(* Logix 5000 Rung export; software revision 16.04 *)

MODULES
   Local : vendor None type None code None
   AFC : vendor None type None code None
END_MODULES

TYPE AFC_ModbusPassThruIn :   // Modbus pass through input
STRUCT
   BID : INT;   // Calculated by ladder logic
   MessagePresent : BOOL;   // Message present in the response block
   Function_BitWrite : BOOL;   // Function bit write
   OverflowError : BOOL;   // Overflow error flag
   ModbusAddress : INT;   // Destination modbus address
   RegisterCount : INT;   // Number of elements associated to command
   ReadData_Word : INT[125];   // Contains received data for word commands
   ReadData_Bit : BOOL[2016];   // Contains received data for bit commands
END_STRUCT
END_TYPE

TYPE AFC_Prove_Config :   // Controls (configuration settings) associated to the prover
STRUCT
   Enable : AFC_Prove_Config_Enable;   // Controls at enable
   Accept : AFC_Prove_Config_Accept;   // Controls at accept
END_STRUCT
END_TYPE

TYPE AFC_Prove_Phase_Bitmap :   // AFC prove phase bitmap
STRUCT
   Not_Selected : BOOL;   // Not selected
   Active : BOOL;   // Active, not counting
   Counting_Past_1st_Switch : BOOL;   // Counting past 1st switch for Udir and forward leg for Bdir)
   Past_2nd_Switch_Fwd_Leg : BOOL;   // Past 2nd switch forward leg (bidirectional only)
   Past_1st_Swith_Ret_Leg : BOOL;   // Past 1st switch return leg (bidirectional only)
   Run_Complete : BOOL;   // Run complete. past 2nd switch.
END_STRUCT
END_TYPE

TYPE AFC :   // Main user defined data type
STRUCT
   Meters : AFC_Meters[16];   // Stores meter process variables, results, analysis (gas) and module profile
   MeterSignals : AFC_Meter_Reset;   // Sets meter signals (write archive, reset accumulator and select stream)
   ModbusGateway : AFC_Modbus;   // Reads and write data between processor and module modbus table
   ModbusMaster : AFC_ModbusMaster;   // Setup modbus master commands to be sent to remote slaves (through Port 3)
   ModbusPassThru : AFC_ModbusPassThru;   // Modbus pass-thru data
   Prove : AFC_Prove;   // Proving implementation (only firmware 2.07.000 or later)
   Flags : AFC_Flag;   // Wallclock update commands
   EnableMeter : AFC_Meter;   // Enable meters (this action can also be performed through AFC Manager)
   DisableMeter : AFC_Meter;   // Disable meters (this action can also be performed through AFC Manager)
   EnableStatus : AFC_Meter;   // Meter current status (0=disabled, 1=enabled)
   Site_Status : AFC_Site_Status;   // Site status
   Site_Alarms : AFC_Site_Alarms;   // Site Alarms
   CycleCounter : INT;   // Reflects current block ID calculated by ladder to be sent to the module
   inputbuffer : INT[250];   // Input buffer contains the complete block to be copied from the module
   outputbuffer : INT[248];   // Output buffer contains data the complete block to be copied to the module
   clockstructure : AFC_Time;   // Stores clock information
   Util : AFC_Util;   // Convenience variables used by ladder logic
END_STRUCT
END_TYPE

TYPE AFC_ModbusGateway :   // Modbus gateway complete data structure
STRUCT
   Config : AFC_ModbusConfig;   // Config data to be entered by the user.
   BOD : INT;   // Block ID automatically generated by ladder
   WriteData : INT[200];   // Contains modbus data written to the module (write commands)
   BID : INT;   // Block ID automatically generated by ladder
   ReadData : INT[200];   // Contains modbus data read from the module (read commands)
END_STRUCT
END_TYPE

TYPE AFC_Meter_Variables :   // Meter process variables from processor to the module.
STRUCT
   BID : INT;   // Block ID associated to meter process variable block (from processor to the module)
   DifferentialGas : AFC_Meter_Differential_Gas_Output;   // Differential meter and gas product
   DifferentialLiquid : AFC_Meter_Differential_Liquid_Output;   // Differential meter and liquid product
   LinearGas : AFC_Meter_Linear_Gas_Output;   // Linear meter and gas product
   LinearLiquid : AFC_Meter_Linear_Liquid_Output;   // Linear meter and liquid product
END_STRUCT
END_TYPE

TYPE AFC_Components_Low :   // Low precision gas component analysis
STRUCT
   C1 : INT;   // Methane
   N2 : INT;   // Nitrogen
   CO2 : INT;   // Carbon dioxide
   C2 : INT;   // Ethane
   C3 : INT;   // Propane
   H20 : INT;   // Water
   H2S : INT;   // Hydrogen sulphide
   H2 : INT;   // Hydrogen
   CO : INT;   // Carbon monoxide
   O2 : INT;   // Oxygen
   IC4 : INT;   // Iso-butane
   NC4 : INT;   // Normal butane
   IC5 : INT;   // Iso-pentane
   NC5 : INT;   // Normal pentane
   C6 : INT;   // Hexane
   C7 : INT;   // Heptane
   C8 : INT;   // Octane
   C9 : INT;   // Nonane
   C10 : INT;   // Decane
   He : INT;   // Helium
   Ar : INT;   // Argon
   NeoC5 : INT;   // Not used
   Ux_User1 : INT;   // Not used
   Uy_User2 : INT;   // Not used
END_STRUCT
END_TYPE

TYPE AFC_Modbus :   // Modbus Gateway data structure. Select the number of commands to be used (1 to 10). O will disable this funcionality.
STRUCT
   CommandCount : INT;   // Defines the number of Modbus Gateway Blocks to be used (1 to 10). Set to 0 to disable the feature.
   Command : AFC_ModbusGateway[10];   // Modbus gateway commands - contains setup and modbus data
END_STRUCT
END_TYPE

TYPE AFC_Status :   // General meter configuration profile
STRUCT
   MeterType : BOOL;   // 0=Differential, 1=Linear
   ProductGroup : BOOL;   // 0=Gas, 1=Liquid
   SelectedStream : INT;   // Selected Stream (1 through 4). Only supported for firmware version 2.05.000 or later
END_STRUCT
END_TYPE

TYPE AFC_Prove_Process :   // Prove process output from processor to the module
STRUCT
   Sequencing : AFC_Prove_Sequencing;   // Prover sequencing
   Temperature : REAL;   // Temperature for Single Probe provers. And Inlet Temperature for Dual Probe Provers.
   Outlet_Temperature : REAL;   // Outlet Temperature for Provers with Dual Probes.
   Switch_Bar_Temperature : REAL;   // Switch bar temperature
   Pressure : REAL;   // Pressure for Single Probe provers. And Inlet Pressure for Dual Probe Provers.
   Outlet_Pressure : REAL;   // Outlet Pressure for Provers with Dual Probes.
   Prover_Density : REAL;   // Prover density
END_STRUCT
END_TYPE

TYPE AFC_Analysis_Status :   // Contains stream configuration information concerning high/low precision.
STRUCT
   Update : BOOL;   // Trigger update of analysis status
   Stream_Precision : SINT[4];   // Stream Precision ( 1 = Low, 2 = High)
   Slot_In_Stream : SINT[4];   // Slot number associated to each stream (0-BASED) Ex: (Slot_In_Stream[0] = 1 means stream 1 is set for slot 2)
   Slot_Precision : SINT[4];   // Precision of each slot (0-BASED) (2=high precision/first slot, 1=low precision,0=high precision/second slot)
END_STRUCT
END_TYPE

TYPE AFC_Meter_Differential_Gas_Output :   // Process Variables for differential meter with gas product
STRUCT
   Temperature : REAL;   // Temperature
   Pressure : REAL;   // Static pressure
   Differential_Pressure : REAL;   // Differential pressure if Primary Input = Differential pressure OR Flow Rate if Primary Input = Flow rate
END_STRUCT
END_TYPE

TYPE AFC_Site_Status :   // Site status bits - contains general information about the module - not meter specific
STRUCT
   AFC_ACTIVE : BOOL;   // AFC active
   Checksum_Alarms : BOOL;   // Checkum alarm active
   reserved2 : BOOL;
   reserved3 : BOOL;
   PLC_HALTED : BOOL;   // PLC in program mode or missing
   Cfg_changed : BOOL;   // Configuration changed
   Powerup : BOOL;   // Module powered up
   ColdStart : BOOL;   // Module performed cold start (BBRAM initialized)
   HardPassword : BOOL;   // Hard password selected
   reserved9 : BOOL;
   reserved10 : BOOL;
   reserved11 : BOOL;
   reserved12 : BOOL;
   reserved13 : BOOL;
   reserved14 : BOOL;
   reserved15 : BOOL;
END_STRUCT
END_TYPE

TYPE AFC_Meter_Linear_Liquid_Output :   // Process Variables for linear meter with liquid product
STRUCT
   Water_Percent : INT;   // Water (%)
   Temperature : REAL;   // Temperature
   Pressure : REAL;   // Pressure
   Meter_Pulses : DINT;   // Meter pulses
   Density : REAL;   // Density
   Pulse_Frequency : REAL;   // Pulse frequency (Hz)
END_STRUCT
END_TYPE

TYPE AFC_Prove_Pulse_Count :   // Values to be supplied at the end of the pass/run
STRUCT
   Meter : DINT;   // Meter pulse count
   Master_Meter : DINT;   // Master meter pulse count
END_STRUCT
END_TYPE

TYPE AFC_Prove_Run_Results :   // Run results of the prove. Copied from the module to the pocessor
STRUCT
   Count_Attempted : INT;   // Run count attempted
   Count_Completed : INT;   // Run count completed
   Count_Selected : INT;   // Run count selected
   Runs_Selected : INT;   // Bit Mapped Runs selected for calculations from completed runs
   New_Meter_Factor : REAL;   // New meter factor
   Change_In_Meter_Factor : REAL;   // Change in meter factor
END_STRUCT
END_TYPE

TYPE AFC_ModbusMasterSwap :   // Modbus master swap words/ swap bytes
STRUCT
   Swap_Words : BOOL;   // Swap words
   Swap_Bytes : BOOL;   // Swap bytes
END_STRUCT
END_TYPE

TYPE AFC_Prove_Config_Enable :   // Prove controls at enable
STRUCT
   Meter_Number : INT;   // Meter number requested (1-16)
   Auto_Accept_Prove : BOOL;   // Auto-accept the prove
   Auto_Continue_Prove : BOOL;   // Auto-continue the prove
END_STRUCT
END_TYPE

TYPE AFC_ModbusMasterIn :   // Modbus master input tag.
STRUCT
   BID : INT;   // Block id associated to modbus master request
   TransactionNumber : INT;   // Transaction number associated to modbus command index
   ErrorCode : INT;   // Error code associated to modbus master command
   Pending : BOOL;   // Pending modbus master command - waiting for modbus response
   ReadData : INT[100];   // Data read fro mremote slave device
END_STRUCT
END_TYPE

TYPE AFC_Prove_Input :   // AFC Prove input block
STRUCT
   Config : AFC_Prove_Input_Config;   // AFC prover input configuration
   Status : AFC_Prove_Status;   // AFC prover status
   Error_Code : INT;   // Prove error code
   Prove_controls_Echo : INT;   // AFC module Echos the state of the Prove Controls
   Requested_Meter_Echo : INT;   // AFC module Echos the Meter number requested
   Requested_Curve_Point_Echo : INT;   // AFC module Echos the requested Curve Point
   Run_Results : AFC_Prove_Run_Results;   // Prove and run results
   Prove_Enabled : BOOL;   // ON if prove is enabled. This flag is coped from inputbuffer[247]
END_STRUCT
END_TYPE

TYPE AFC_Util :   // Used for internal ladder logic usage. These values must not be changed by user application.
STRUCT
   MeterIndex1 : INT;   // Meter index for process variable calculation
   Offset1 : INT;   // Offset for meter process calculation
   MeterIndex2 : INT;   // Meter index for calculation results
   Offset2 : INT;   // Offset for calculation results
   SignalsTimer : TIMER;   // Signals timer
   IndexOut : INT;   // Index output
   IndexIn : INT;   // Index input
   CycleCounterRollover : INT;   // Rollover value for cycle counter for block ID calculation
   LongCount : INT;   // Long count for modbus master command
   LastRegularBlockID : INT;   // Rollover block ID
   Current_meter : SINT;   // Current meter number analysis update
   MaskedStream : INT;   // Masked stream
   AnalysisMeterNumber : INT;   // Analysis meter number
   AnalysisBID : INT;   // Analysis block ID
   AnalysisStreamMasked : INT;   // Analysis stream masked information
   v206orLater : INT;   // indicates if the meter is 2.06 or later so the module supports high precision analysis
   AnalysisHighPrecisionBOD : INT;   // Analysis high precision number
   Firmware_Version : SINT[2];   // Firmware version number
   Firmware_Revision : INT;   // firmware revision number
   AnalysisHMeter : INT;   // Meter associated to molar high precision
   SlotPrecision : SINT[4];   // Slot precision number for stream precision calculation
   SlotInStream : DINT[4];   // Slot number for stream X
   PowerUp_HighAnalysis : BOOL;   // Request high analysis block upon power up
   Meter_HighAnalysis : INT;   // Meter number for high precision analysis
   TempSlotInStream : SINT;   // Used to calculate stream precision based on slot precision
   AnalysisHighPrecisionBID : INT[16];   // High precision block ID
   AnalysisHighPrecisionBID_Update : INT;   // molar block id update
   Reinitialize_Timer : TIMER;   // Timer to initialize block ID if freezes
   Prover_Phase : INT;   // Prover phase integer word to assemble all bits
   Prover_Signals : INT;   // Prover signals integer word to assemble all bits
   Prover_Controls : INT;   // Prover control word to assemble all bits
END_STRUCT
END_TYPE

TYPE AFC_Time :   // AFC time format used for walclock update
STRUCT
   Year : DINT;   // Year
   Month : DINT;   // Month
   Day : DINT;   // Day
   Hour : DINT;   // Hour
   Minute : DINT;   // Minute
   second : DINT;   // Seconds
   msec : DINT;   // Milliseconds
END_STRUCT
END_TYPE

TYPE AFC_ModbusPassThru :   // AFC modbus pass through controller tag
STRUCT
   Output : AFC_ModbusPassThruOut;   // Values to be transferred from processor to the module
   Input : AFC_ModbusPassThruIn;   // Values to be transferred from module to processor
END_STRUCT
END_TYPE

TYPE AFC_Meter_Results :   // AFC meter results calculated by the module to the processor
STRUCT
   BID : INT;   // Block ID associated to calculation results
   Alarms : INT;   // Meter alarms
   DifferentialGas : AFC_Meter_Differential_Gas_Input;   // Differential meter / product gas
   DifferentialLiquid : AFC_Meter_Differential_Liquid_Input;   // Differential meter / product liquid
   LinearGas : AFC_Meter_Linear_Gas_Input;   // Linear meter / product gas
   LinearLiquid : AFC_Meter_Linear_Liquid_Input;   // Linear meter / product liquid
END_STRUCT
END_TYPE

TYPE AFC_Prove_Config_Accept :   // Prove controls at accept. If auto-accept is selected must be available at enable
STRUCT
   Requested_Interpolation_Point : INT;   // Requested interpolation point (0 nearest)
   Apply_MF_Change_All_Streams : BOOL;   // Apply change in meter factor to all streams
   Apply_MF_Change_Curve : BOOL;   // Apply change in meter factor to all curve points
   Apply_New_MF : BOOL;   // CApply new meter factor
END_STRUCT
END_TYPE

TYPE AFC_Meter_Signals :   // Meter signals options
STRUCT
   Sel_Stream1 : BOOL;   // Set to 1 to select stream 1
   Sel_Stream2 : BOOL;   // Set to 1 to select stream 2
   Sel_Stream3 : BOOL;   // Set to 1 to select stream 3
   Sel_Stream4 : BOOL;   // Set to 1 to select stream 4
   Res_Acc1 : BOOL;   // Set to 1 to reset resettable accumulator 1
   Res_Acc2 : BOOL;   // Set to 1 to reset resettable accumulator 2
   Res_Acc3 : BOOL;   // Set to 1 to reset resettable accumulator 3
   Res_Acc4 : BOOL;   // Set to 1 to reset resettable accumulator 4
   Wr_Daily_Archive : BOOL;   // Set to 1 to write daily archive
   Wr_Hrly_Archive : BOOL;   // Set to 1 to write hourly archive
END_STRUCT
END_TYPE

TYPE AFC_ModbusMasterDataType :   // Modbus master data type selection
STRUCT
   Bit : BOOL;   // bit type
   Word : BOOL;   // word type (16-bit)
   Long : BOOL;   // long integer (32-bit)
   LongRemote : BOOL;   // long integer (32-bit)
END_STRUCT
END_TYPE

TYPE AFC_Prove_Status :   // Status of the prove (returned from the module to the processor)
STRUCT
   Prove_Accepted : BOOL;   // Prove was accepted
   Meter_Factor_Applied : BOOL;   // Meter factor was applied
   MF_Applied_To_Curve : BOOL;   // Meter factor was applied to all points in the curve
   MF_Applied_To_Streams : BOOL;   // Meter factor was applied to all streams
   Prove_Rejected_By_Command : BOOL;   // Prove was rejected by command
   Prove_Rejected_No_Runs : BOOL;   // Prove was rejected - empty prove (no runs)
   Prove_Rejected_Divide_By_0 : BOOL;   // Prove was rejected - divide by 0
   Prove_Enabled : BOOL;   // Prove is enabled
   Proving_Run_In_Progress : BOOL;   // Proving run is in progress
   Prove_Rejected_Abort : BOOL;   // Prove rejected: abort
   Prove_Paused : BOOL;   // Prove is paused
   Run_Cancelled : BOOL;   // Run Is cancelled
   Run_Timed_Out : BOOL;   // Run timed out
END_STRUCT
END_TYPE

TYPE AFC_Prove :   // Implements prove funcionality. Supported only for firmware version 2.07 or later.
STRUCT
   Output : AFC_Prove_Output;   // Prover output block to the module
   Input : AFC_Prove_Input;   // Prover input block from the module
END_STRUCT
END_TYPE

TYPE AFC_Meter_Differential_Liquid_Output :   // Process Variables for differential meter with liquid product
STRUCT
   Water_Percent : INT;   // Water %
   Temperature : REAL;   // Temperature
   Pressure : REAL;   // Static Pressure
   Differential_Pressure : REAL;   // Differential pressure if Primary Input = Differential pressure OR Flow Rate if Primary Input = Flow rate
   Density : REAL;   // Density
END_STRUCT
END_TYPE

TYPE AFC_Meter_Differential_Liquid_Input :   // Calculation Results for differential meter with lliquid product
STRUCT
   Net_Accumulator : DINT;   // Net accumulator
   Net_Flowrate : REAL;   // Net flow rate
   Gross_Accumulator : DINT;   // Gross acumulator
   Gross_Standard_Accumulator : DINT;   // Gross standard accumulator
   Mass_Accumulator : DINT;   // Mass accumulator
END_STRUCT
END_TYPE

TYPE AFC_Analysis_Low :   // Low precision (16-bit word) Gas Analysis support.
STRUCT
   EnableContinuous : BOOL;   // Set to ON to update the low precision molar analysis. The data will be updated continuously while the molar analysis is updated.
   Stream : INT;   // Select stream for molar analysis (low precision) update. Valid range is 0 (active) and 1 to 4.
   Components : AFC_Components_Low;   // Gas components in low precision format (16-bit word)
END_STRUCT
END_TYPE

TYPE AFC_Meter_Differential_Gas_Input :   // Calculation results for differential meter with gas product
STRUCT
   Net_Accumulator : DINT;   // Net accumulator
   Net_Flowrate : REAL;   // Net flow rate
   Gross_Flowrate : REAL;   // Gross flow rate
   Fpv : REAL;   // Super compressibility
   Cprime : REAL;   // Cprime
END_STRUCT
END_TYPE

TYPE AFC_Prove_Input_Config :   // Prove input block results - prover configuration
STRUCT
   Type : INT;   // Prover type
   Options : INT;   // Prover options
   Runs_Per_Prove_Total : INT;   // Total runs per prove
   Runs_Per_Prove_Selected : INT;   // Selected runs per prove
   Max_Runs_before_Abort : INT;   // Max total runs before abort
   Short_Passes_Per_Run : INT;   // Short passes per run if bidir = 2 , else 0
END_STRUCT
END_TYPE

TYPE AFC_Flag :   // Flags contains status information updated by ladder and also trigger bits for clock update
STRUCT
   AFC_Stopped : BOOL;   // Indicates that the module has sent a new input block to be processed by ladder - UPDATED BY LADDER
   AFC_InputSequenceNum : INT;   // Meter number (0 -15) associated to blocks 1-16. Used to update "Profile" (meter type and product group.) UPDATED BY LADDER
   AFC_Set_Clock : BOOL;   // Set to 1 to update module wallclock (using processor as a source) UPDATED BY USER
   plc_set_clock : BOOL;   // Set to 1 to set processor wallclock UPDATED BY USER
END_STRUCT
END_TYPE

TYPE AFC_Meter_Analysis :   // Meter analysis components. Allows the processor to update molar analysis for low precision and high precision streams.
STRUCT
   Low_Precision : AFC_Analysis_Low;   // Low precision gas components (16-bit word per component)
   High_Precision : AFC_Analysis_High;   // High precision gas components (floating point per component). Only supported for firmware version 2.07.000 or later
   Status : AFC_Analysis_Status;   // Stream analysis status - contains stream and slot configuration data
END_STRUCT
END_TYPE

TYPE AFC_ModbusMasterElement :   // Modbus master controller tag. Requires port 3 to be configured as a modbus master device.
STRUCT
   Output : AFC_ModbusMasterOut;   // From processor to the module
   Input : AFC_ModbusMasterIn;   // From module to the processor
END_STRUCT
END_TYPE

TYPE AFC_Analysis_High :   // High precision (floating point) Gas Analysis support. This feature is only supported for firmware version 2.07.000 or later
STRUCT
   EnableOnce : BOOL;   // Set to ON to request the high precision analysis update one time. It automatically resets to 0 after the request.
   Stream : INT;   // Stream number. Range is 0 (active) and 1 to 4.
   Components : AFC_Components_High;   // AFC High Precision Molar Analysis (floating point)
END_STRUCT
END_TYPE

TYPE AFC_Site_Alarms :   // Indicates if a meter has any alarms
STRUCT
   Meter1 : BOOL;   // Meter in alarm
   Meter2 : BOOL;   // Meter in alarm
   Meter3 : BOOL;   // Meter in alarm
   Meter4 : BOOL;   // Meter in alarm
   Meter5 : BOOL;   // Meter in alarm
   Meter6 : BOOL;   // Meter in alarm
   Meter7 : BOOL;   // Meter in alarm
   Meter8 : BOOL;   // Meter in alarm
   Meter9 : BOOL;   // Meter in alarm
   Meter10 : BOOL;   // Meter in alarm
   Meter11 : BOOL;   // Meter in alarm
   Meter12 : BOOL;   // Meter in alarm
   Meter13 : BOOL;   // Meter in alarm
   Meter14 : BOOL;   // Meter in alarm
   Meter15 : BOOL;   // Meter in alarm
   Meter16 : BOOL;   // Meter in alarm
END_STRUCT
END_TYPE

TYPE AFC_ModbusPassThruOut :   // AFC Modbus pass through output block fro mprocessor to the module
STRUCT
   BOD : INT;   // Automatically calculated by sample ladder
   Enable : BOOL;   // Set to 1 to enable pass-thru funcionality (requires AFC Manager setting)
END_STRUCT
END_TYPE

TYPE AFC_Components_High :   // High precision gas component analysis (only supported version 2.07.000)
STRUCT
   C1 : REAL;   // Methane
   N2 : REAL;   // Nitrogen
   CO2 : REAL;   // Carbon Dioxide
   C2 : REAL;   // Ethane
   C3 : REAL;   // Propane
   H20 : REAL;   // Water
   H2S : REAL;   // Hydrogen Sulphide
   H2 : REAL;   // Hydrogen
   CO : REAL;   // Carbon Monoxide
   O2 : REAL;   // Oxygen
   IC4 : REAL;   // Iso-butane
   NC4 : REAL;   // Normal Butane
   IC5 : REAL;   // Iso-pentane
   NC5 : REAL;   // Normal-pentane
   C6 : REAL;   // Hexane
   C7 : REAL;   // Heptane
   C8 : REAL;   // Octane
   C9 : REAL;   // Nonane
   C10 : REAL;   // Decane
   He : REAL;   // Helium
   Ar : REAL;   // Argon
   NeoC5 : REAL;   // Not Used
   Ux_User1 : REAL;   // Not Used
   Uy_User2 : REAL;   // Not Used
END_STRUCT
END_TYPE

TYPE AFC_Prove_Signals :   // Contains the proving signals that will trigger specific tasks from the module
STRUCT
   EnableProve : BOOL;   // Enables the prove
   AcceptProve : BOOL;   // Accepts the prove
   RejectProve : BOOL;   // Reject the prove
   RunStart : BOOL;   // Starts the run
   RunComplete : BOOL;   // Flags that the run is complete
   RunCancel : BOOL;   // Cancels the run
   RunDelete : BOOL;   // Deletes the run
   PassComplete : BOOL;   // Flag that the pass is complete
   PauseProve : BOOL;   // Pauses the Proving Process
   AbortProve : BOOL;   // Aborts the prove
END_STRUCT
END_TYPE

TYPE AFC_Meter_Reset :   // Meter signals to request for reset accumulator, select stream and write archives.
STRUCT
   Enable : BOOL;   // Enable meter signal request. UPDATED BY USER
   BID : INT;   // Block ID for meter signal request. UPDATED BY LOGIC
   Meter : INT;   // Meter number (1-16) associated to signal request UPDATED BY USER
   Action : INT;   // Action word built from Signal bits (UPDATED by USER)
   Signals : AFC_Meter_Signals;   // Signals request bits
   ResetOnce : BOOL;   // Request signal update once
   LastBlockID : INT;   // Last block ID associated to signals request
END_STRUCT
END_TYPE

TYPE AFC_ModbusMasterOut :   // Modbus master request from processor to the module
STRUCT
   Config : AFC_ModbusMasterConfig;   // Modbus master command configuration settings
   TransactionNumber : INT;   // Transaction number used to keep track of diffeernt commands (echoed back in response)
   BOD : INT;   // Block output ID
   WriteData : INT[100];   // Write data associated to the write command
END_STRUCT
END_TYPE

TYPE AFC_Meters :   // Main meter data structure. Contains process variables, calculation results, gas analysis, profile update
STRUCT
   Variables : AFC_Meter_Variables;   // Input process variables to be transferred to the module
   Results : AFC_Meter_Results;   // Calculation results transferred from the module
   Analysis : AFC_Meter_Analysis;   // Molar Analysis data to be transferred to the module (only for gas products with online gas chromatograph applications)
   Profile : AFC_Status;   // Module profile (meter type/product group) transfered from the module
END_STRUCT
END_TYPE

TYPE AFC_ModbusMaster :   // Modbus master operation. Port 3 must be configured as modbus master through AFC Manager to use this feature.
STRUCT
   Enable : BOOL;   // Enable the modbus master funcionality
   CommandIndex : INT;   // Selects which command index will be executed
   Command : AFC_ModbusMasterElement[10];   // Each command contains a specific modbus request to be sent out of the port
END_STRUCT
END_TYPE

TYPE AFC_Meter :   // Used for meter enable and disable tags
STRUCT
   Meter1 : BOOL;   // Meter 1
   Meter2 : BOOL;   // Meter 2
   Meter3 : BOOL;   // Meter 3
   Meter4 : BOOL;   // Meter 4
   Meter5 : BOOL;   // Meter 5
   Meter6 : BOOL;   // Meter 6
   Meter7 : BOOL;   // Meter 7
   Meter8 : BOOL;   // Meter 8
   Meter9 : BOOL;   // Meter 9
   Meter10 : BOOL;   // Meter 10
   Meter11 : BOOL;   // Meter 11
   Meter12 : BOOL;   // Meter 12
   Meter13 : BOOL;   // Meter 13
   Meter14 : BOOL;   // Meter 14
   Meter15 : BOOL;   // Meter 15
   Meter16 : BOOL;   // Meter 16
END_STRUCT
END_TYPE

TYPE AFC_Meter_Linear_Gas_Output :   // Process Variables for linear meter with gas product
STRUCT
   Temperature : REAL;   // Temperature
   Pressure : REAL;   // Pressure
   Meter_Pulses : DINT;   // Pulse count
   Pulse_Frequency : REAL;   // Pulse Frequency (Hz)
END_STRUCT
END_TYPE

TYPE AFC_Meter_Linear_Liquid_Input :   // Calculation Results for linear meter with liquid product
STRUCT
   Net_Accumulator : DINT;   // Net accumulator
   Net_Flowrate : REAL;   // Net flow rate
   Gross_Accumulator : DINT;   // Gross accumulator
   Gross_Standard_Accumulator : DINT;   // Gross standard accumulator
   Mass_Accumulator : DINT;   // Mass accumulator
END_STRUCT
END_TYPE

TYPE AFC_ModbusConfig :   // Modbus gateway configuration options
STRUCT
   Enable : BOOL;   // Set to 1 to enable modbus gateway command (0=disable)
   StartRegister : INT;   // Start modbus address
   RegisterCount : INT;   // Word count (200 max)
   FunctionType_Write : BOOL;   // 0 = read command, 1 = write command
   RegisterType_Input : BOOL;   // 0 = holding register, 1 = input register
   SlaveType_Virtual : BOOL;   // 0 = primary slave, 1 = virtual slave
END_STRUCT
END_TYPE

TYPE AFC_ModbusMasterConfig :   // Modbus master command settings
STRUCT
   Enable : BOOL;   // Set to 1 to enable command (0=disable)
   FunctionType_Write : BOOL;   // Set to 1 to select write command (0=read command)
   RegisterBank_Input : BOOL;   // Set to 1 to select input register (0=holding register)
   DataType : AFC_ModbusMasterDataType;   // Select data type format
   SwapOption : AFC_ModbusMasterSwap;   // Select byte and word swap (1 = swap, 0 = no swap)
   Type_Swap : INT;   // This value is calculated by ladder logic and must not be modified by user
   SlaveAddress : INT;   // Modbus slave address of remote device
   ModbusAddress : INT;   // Modbus data address on remote slave
   ElementCount : INT;   // Number of data elements (125 words)
END_STRUCT
END_TYPE

TYPE AFC_Prove_Sequencing :   // AFC prove sequencing tag for phase selection and ball positioning
STRUCT
   Phase : AFC_Prove_Phase_Bitmap;   // AFC phase sequencing
   Ball_Position_Ready : BOOL;   // Ball position: Ready (Udir & Bdir only; fwd leg Bdir)
   Ball_Position_Sealed : BOOL;   // Ball position: Sealed (Udir & Bdir only; fwd leg Bdir)
   Ball_Position_Ready_Bwd_Leg : BOOL;   // Ball position: Ready bwd leg (Bdir only)
   Ball_Position_Sealed_Bwd_Leg : BOOL;   // Ball position: Sealed bwd leg (Bdir only)
END_STRUCT
END_TYPE

TYPE AFC_Prove_Output :   // AFC Prove output block
STRUCT
   Process : AFC_Prove_Process;   // Process Variables
   Signals : AFC_Prove_Signals;   // AFC Prove Signals (triggers the proving update)
   Config : AFC_Prove_Config;   // AFC Prove Control (configuration settings)
   Pulse_Counts : AFC_Prove_Pulse_Count;   // Pulse counts to be updated at the end of the run/pass
END_STRUCT
END_TYPE

TYPE AFC_Meter_Linear_Gas_Input :   // Calculation Results for linear meter with gas product
STRUCT
   Net_Accumulator : DINT;   // Net accumulator
   Net_Flowrate : REAL;   // Net flow rate
   Gross_Flowrate : REAL;   // Gross flow rate
   Fpv : REAL;   // Supercompressibility
   CPrime : REAL;   // CPrime
END_STRUCT
END_TYPE

ADD_ON_INSTRUCTION AOI56AFC   (* revision 1.3, vendor ProSoft Technology Inc, ExecutePrescan *)
// MVI56-AFC Add-On Instruction
// Revision note:
// - Supports proving and high analysis (v2.07.000)
// - Fixes minor fault to CLX
// - Copies CPrime for Linear/Gas meter
// Help:
// v1.3 Update Modbus Gateway Read Function.
VAR_IN_OUT
   Connection_Input : INT[250]; {required}
   Connection_Output : INT[248]; {required}
   AFC56 : AFC; {required}
END_VAR
VAR
   MJFAULTS : DINT[12];
END_VAR

ROUTINE Logic   (* ladder *)
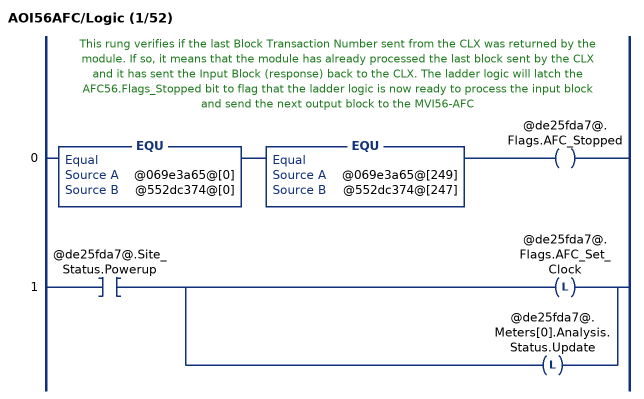
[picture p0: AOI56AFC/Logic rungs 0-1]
   // This rung verifies if the last Block Transaction Number sent from the CLX was returned by the module. If so, it means that the module has already processed the last block sent by the CLX and it has sent the Input Block (response) back to the CLX. The ladder logic will latch the AFC56.Flags_Stopped bit to flag that the ladder logic is now ready to process the input block and send the next output block to the MVI56-AFC
   0: EQU(@069e3a65@[0],@552dc374@[0])EQU(@069e3a65@[249],@552dc374@[247])OTE(@de25fda7@.Flags.AFC_Stopped);
   1: XIC(@de25fda7@.Site_Status.Powerup)[OTL(@de25fda7@.Flags.AFC_Set_Clock) ,OTL(@de25fda7@.Meters[0].Analysis.Status.Update) ];
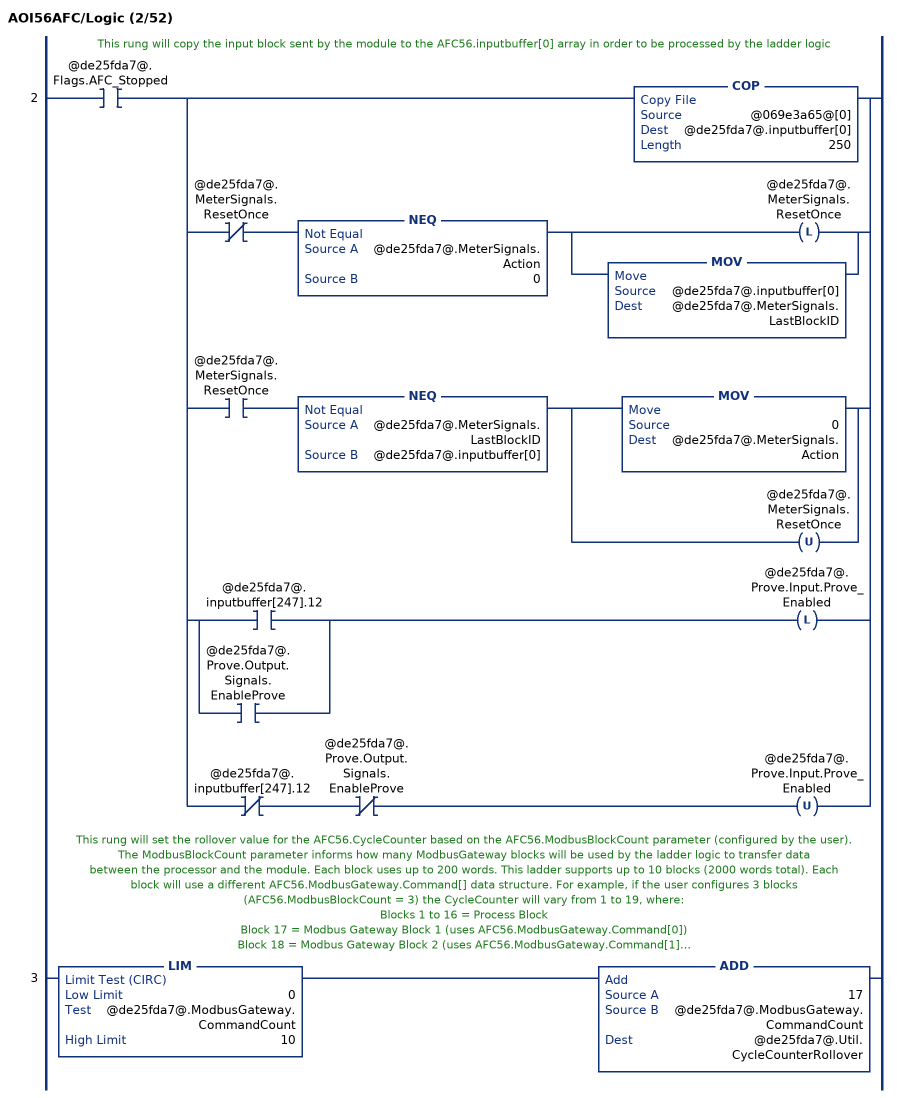
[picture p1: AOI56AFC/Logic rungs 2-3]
   // This rung will copy the input block sent by the module to the AFC56.inputbuffer[0] array in order to be processed by the ladder logic
   2: XIC(@de25fda7@.Flags.AFC_Stopped)[COP(@069e3a65@[0],@de25fda7@.inputbuffer[0],250) ,XIO(@de25fda7@.MeterSignals.ResetOnce) NEQ(@de25fda7@.MeterSignals.Action,0) [OTL(@de25fda7@.MeterSignals.ResetOnce) ,MOV(@de25fda7@.inputbuffer[0],@de25fda7@.MeterSignals.LastBlockID) ] ,XIC(@de25fda7@.MeterSignals.ResetOnce) NEQ(@de25fda7@.MeterSignals.LastBlockID,@de25fda7@.inputbuffer[0]) [MOV(0,@de25fda7@.MeterSignals.Action) ,OTU(@de25fda7@.MeterSignals.ResetOnce) ] ,[XIC(@de25fda7@.inputbuffer[247].12) ,XIC(@de25fda7@.Prove.Output.Signals.EnableProve) ] OTL(@de25fda7@.Prove.Input.Prove_Enabled) ,XIO(@de25fda7@.inputbuffer[247].12) XIO(@de25fda7@.Prove.Output.Signals.EnableProve) OTU(@de25fda7@.Prove.Input.Prove_Enabled) ];
   // This rung will set the rollover value for the AFC56.CycleCounter based on the AFC56.ModbusBlockCount parameter (configured by the user). The ModbusBlockCount parameter informs how many ModbusGateway blocks will be used by the ladder logic to transfer data
   // between the processor and the module. Each block uses up to 200 words. This ladder supports up to 10 blocks (2000 words total). Each block will use a different AFC56.ModbusGateway.Command[] data structure. For example, if the user configures 3 blocks (AFC56.ModbusBlockCount = 3) the CycleCounter will vary from 1 to 19, where:
   // Blocks 1 to 16 = Process Block
   // Block 17 = Modbus Gateway Block 1 (uses AFC56.ModbusGateway.Command[0])
   // Block 18 = Modbus Gateway Block 2 (uses AFC56.ModbusGateway.Command[1])
   // Block 19 = Modbus Gateway Block 3 (uses AFC56.ModbusGateway.Command[2])
   3: LIM(0,@de25fda7@.ModbusGateway.CommandCount,10)ADD(17,@de25fda7@.ModbusGateway.CommandCount,@de25fda7@.Util.CycleCounterRollover);
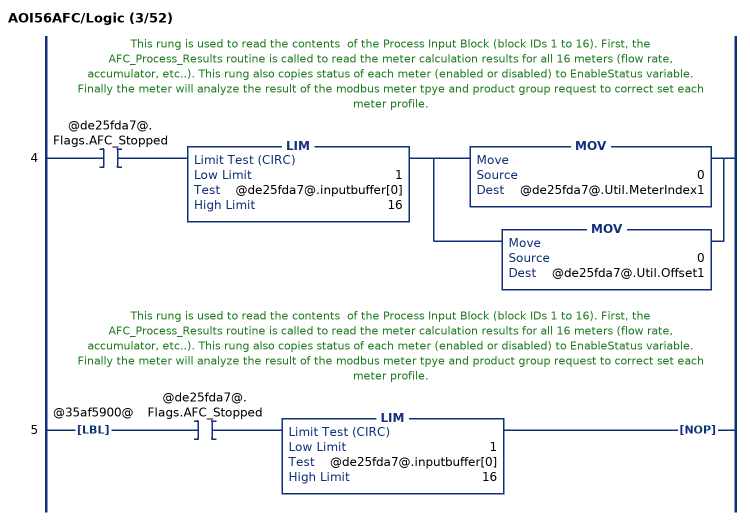
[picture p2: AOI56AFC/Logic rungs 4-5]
   // This rung is used to read the contents  of the Process Input Block (block IDs 1 to 16). First, the AFC_Process_Results routine is called to read the meter calculation results for all 16 meters (flow rate, accumulator, etc..). This rung also copies status of each meter (enabled or disabled) to EnableStatus variable.
   // Finally the meter will analyze the result of the modbus meter tpye and product group request to correct set each meter profile.
   4: XIC(@de25fda7@.Flags.AFC_Stopped)LIM(1,@de25fda7@.inputbuffer[0],16)[MOV(0,@de25fda7@.Util.MeterIndex1) ,MOV(0,@de25fda7@.Util.Offset1) ];
   // This rung is used to read the contents  of the Process Input Block (block IDs 1 to 16). First, the AFC_Process_Results routine is called to read the meter calculation results for all 16 meters (flow rate, accumulator, etc..). This rung also copies status of each meter (enabled or disabled) to EnableStatus variable.
   // Finally the meter will analyze the result of the modbus meter tpye and product group request to correct set each meter profile.
   5: LBL(@35af5900@)XIC(@de25fda7@.Flags.AFC_Stopped)LIM(1,@de25fda7@.inputbuffer[0],16)NOP();
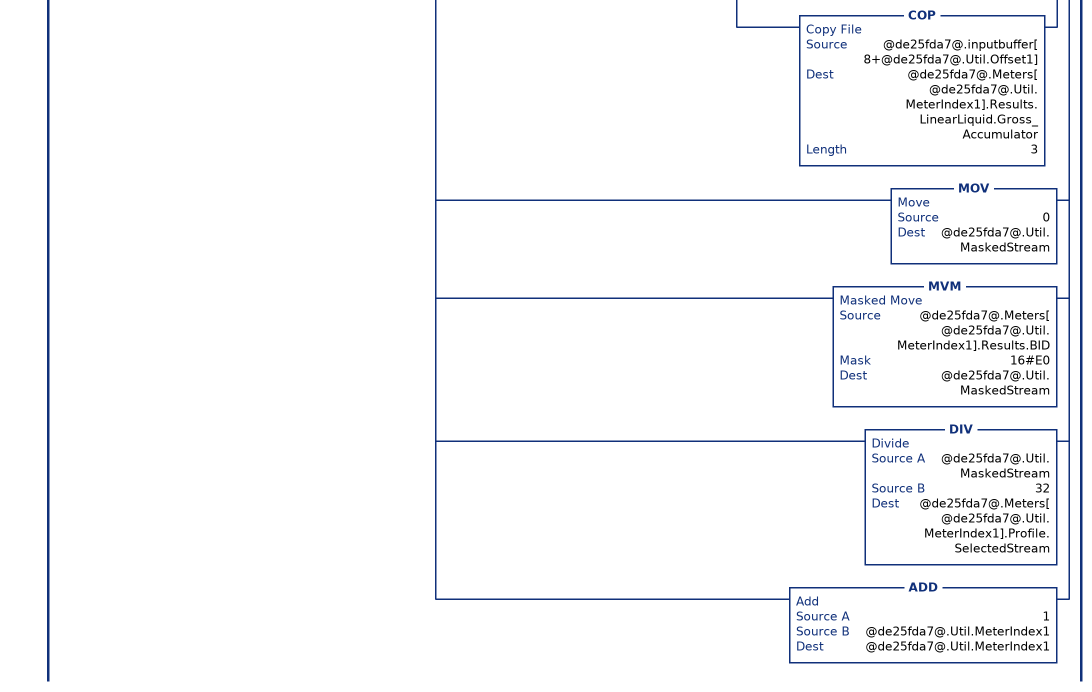
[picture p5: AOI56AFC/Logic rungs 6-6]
   // This rung is used to read the contents  of the Process Input Block (block IDs 1 to 16). First, the AFC_Process_Results routine is called to read the meter calculation results for all 16 meters (flow rate, accumulator, etc..). This rung also copies status of each meter (enabled or disabled) to EnableStatus variable.
   // Finally the meter will analyze the result of the modbus meter tpye and product group request to correct set each meter profile.
   6: XIC(@de25fda7@.Flags.AFC_Stopped)LIM(1,@de25fda7@.inputbuffer[0],16)[CPT(@de25fda7@.Util.Offset1,@de25fda7@.Util.MeterIndex1*12) ,MOV(@de25fda7@.inputbuffer[2+@de25fda7@.Util.Offset1],@de25fda7@.Meters[@de25fda7@.Util.MeterIndex1].Results.BID) ,MOV(@de25fda7@.inputbuffer[3+@de25fda7@.Util.Offset1],@de25fda7@.Meters[@de25fda7@.Util.MeterIndex1].Results.Alarms) ,XIO(@de25fda7@.Meters[@de25fda7@.Util.MeterIndex1].Profile.MeterType) XIO(@de25fda7@.Meters[@de25fda7@.Util.MeterIndex1].Profile.ProductGroup) [COP(@de25fda7@.inputbuffer[4+@de25fda7@.Util.Offset1],@de25fda7@.Meters[@de25fda7@.Util.MeterIndex1].Results.DifferentialGas.Net_Accumulator,1) ,COP(@de25fda7@.inputbuffer[6+@de25fda7@.Util.Offset1],@de25fda7@.Meters[@de25fda7@.Util.MeterIndex1].Results.DifferentialGas.Net_Flowrate,4) ] ,XIO(@de25fda7@.Meters[@de25fda7@.Util.MeterIndex1].Profile.MeterType) XIC(@de25fda7@.Meters[@de25fda7@.Util.MeterIndex1].Profile.ProductGroup) [COP(@de25fda7@.inputbuffer[4+@de25fda7@.Util.Offset1],@de25fda7@.Meters[@de25fda7@.Util.MeterIndex1].Results.DifferentialLiquid.Net_Accumulator,1) ,COP(@de25fda7@.inputbuffer[6+@de25fda7@.Util.Offset1],@de25fda7@.Meters[@de25fda7@.Util.MeterIndex1].Results.DifferentialLiquid.Net_Flowrate,1) ,COP(@de25fda7@.inputbuffer[8+@de25fda7@.Util.Offset1],@de25fda7@.Meters[@de25fda7@.Util.MeterIndex1].Results.DifferentialLiquid.Gross_Accumulator,3) ] ,XIC(@de25fda7@.Meters[@de25fda7@.Util.MeterIndex1].Profile.MeterType) XIO(@de25fda7@.Meters[@de25fda7@.Util.MeterIndex1].Profile.ProductGroup) [COP(@de25fda7@.inputbuffer[4+@de25fda7@.Util.Offset1],@de25fda7@.Meters[@de25fda7@.Util.MeterIndex1].Results.LinearGas.Net_Accumulator,1) ,COP(@de25fda7@.inputbuffer[6+@de25fda7@.Util.Offset1],@de25fda7@.Meters[@de25fda7@.Util.MeterIndex1].Results.LinearGas.Net_Flowrate,4) ] ,XIC(@de25fda7@.Meters[@de25fda7@.Util.MeterIndex1].Profile.MeterType) XIC(@de25fda7@.Meters[@de25fda7@.Util.MeterIndex1].Profile.ProductGroup) [COP(@de25fda7@.inputbuffer[4+@de25fda7@.Util.Offset1],@de25fda7@.Meters[@de25fda7@.Util.MeterIndex1].Results.LinearLiquid.Net_Accumulator,1) ,COP(@de25fda7@.inputbuffer[6+@de25fda7@.Util.Offset1],@de25fda7@.Meters[@de25fda7@.Util.MeterIndex1].Results.LinearLiquid.Net_Flowrate,1) ,COP(@de25fda7@.inputbuffer[8+@de25fda7@.Util.Offset1],@de25fda7@.Meters[@de25fda7@.Util.MeterIndex1].Results.LinearLiquid.Gross_Accumulator,3) ] ,[MOV(0,@de25fda7@.Util.MaskedStream) ,MVM(@de25fda7@.Meters[@de25fda7@.Util.MeterIndex1].Results.BID,16#E0,@de25fda7@.Util.MaskedStream) ,DIV(@de25fda7@.Util.MaskedStream,32,@de25fda7@.Meters[@de25fda7@.Util.MeterIndex1].Profile.SelectedStream) ] ,ADD(1,@de25fda7@.Util.MeterIndex1,@de25fda7@.Util.MeterIndex1) ];
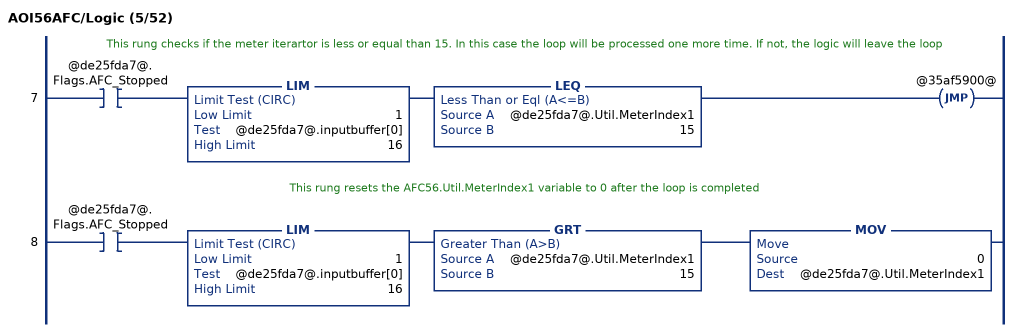
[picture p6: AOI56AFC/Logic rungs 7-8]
   // This rung checks if the meter iterartor is less or equal than 15. In this case the loop will be processed one more time. If not, the logic will leave the loop
   7: XIC(@de25fda7@.Flags.AFC_Stopped)LIM(1,@de25fda7@.inputbuffer[0],16)LEQ(@de25fda7@.Util.MeterIndex1,15)JMP(@35af5900@);
   // This rung resets the AFC56.Util.MeterIndex1 variable to 0 after the loop is completed
   8: XIC(@de25fda7@.Flags.AFC_Stopped)LIM(1,@de25fda7@.inputbuffer[0],16)GRT(@de25fda7@.Util.MeterIndex1,15)MOV(0,@de25fda7@.Util.MeterIndex1);
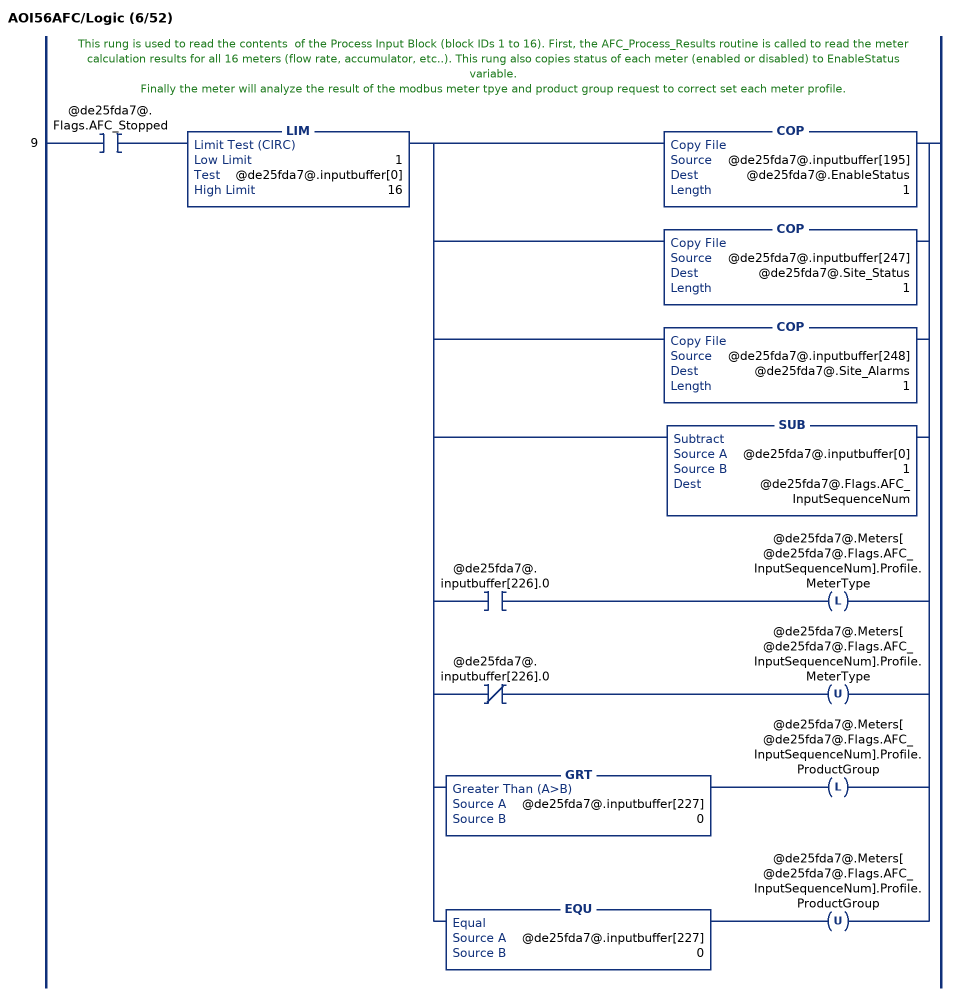
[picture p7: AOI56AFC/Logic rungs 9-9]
   // This rung is used to read the contents  of the Process Input Block (block IDs 1 to 16). First, the AFC_Process_Results routine is called to read the meter calculation results for all 16 meters (flow rate, accumulator, etc..). This rung also copies status of each meter (enabled or disabled) to EnableStatus variable.
   // Finally the meter will analyze the result of the modbus meter tpye and product group request to correct set each meter profile.
   9: XIC(@de25fda7@.Flags.AFC_Stopped)LIM(1,@de25fda7@.inputbuffer[0],16)[COP(@de25fda7@.inputbuffer[195],@de25fda7@.EnableStatus,1) ,COP(@de25fda7@.inputbuffer[247],@de25fda7@.Site_Status,1) ,COP(@de25fda7@.inputbuffer[248],@de25fda7@.Site_Alarms,1) ,SUB(@de25fda7@.inputbuffer[0],1,@de25fda7@.Flags.AFC_InputSequenceNum) ,XIC(@de25fda7@.inputbuffer[226].0) OTL(@de25fda7@.Meters[@de25fda7@.Flags.AFC_InputSequenceNum].Profile.MeterType) ,XIO(@de25fda7@.inputbuffer[226].0) OTU(@de25fda7@.Meters[@de25fda7@.Flags.AFC_InputSequenceNum].Profile.MeterType) ,GRT(@de25fda7@.inputbuffer[227],0) OTL(@de25fda7@.Meters[@de25fda7@.Flags.AFC_InputSequenceNum].Profile.ProductGroup) ,EQU(@de25fda7@.inputbuffer[227],0) OTU(@de25fda7@.Meters[@de25fda7@.Flags.AFC_InputSequenceNum].Profile.ProductGroup) ];
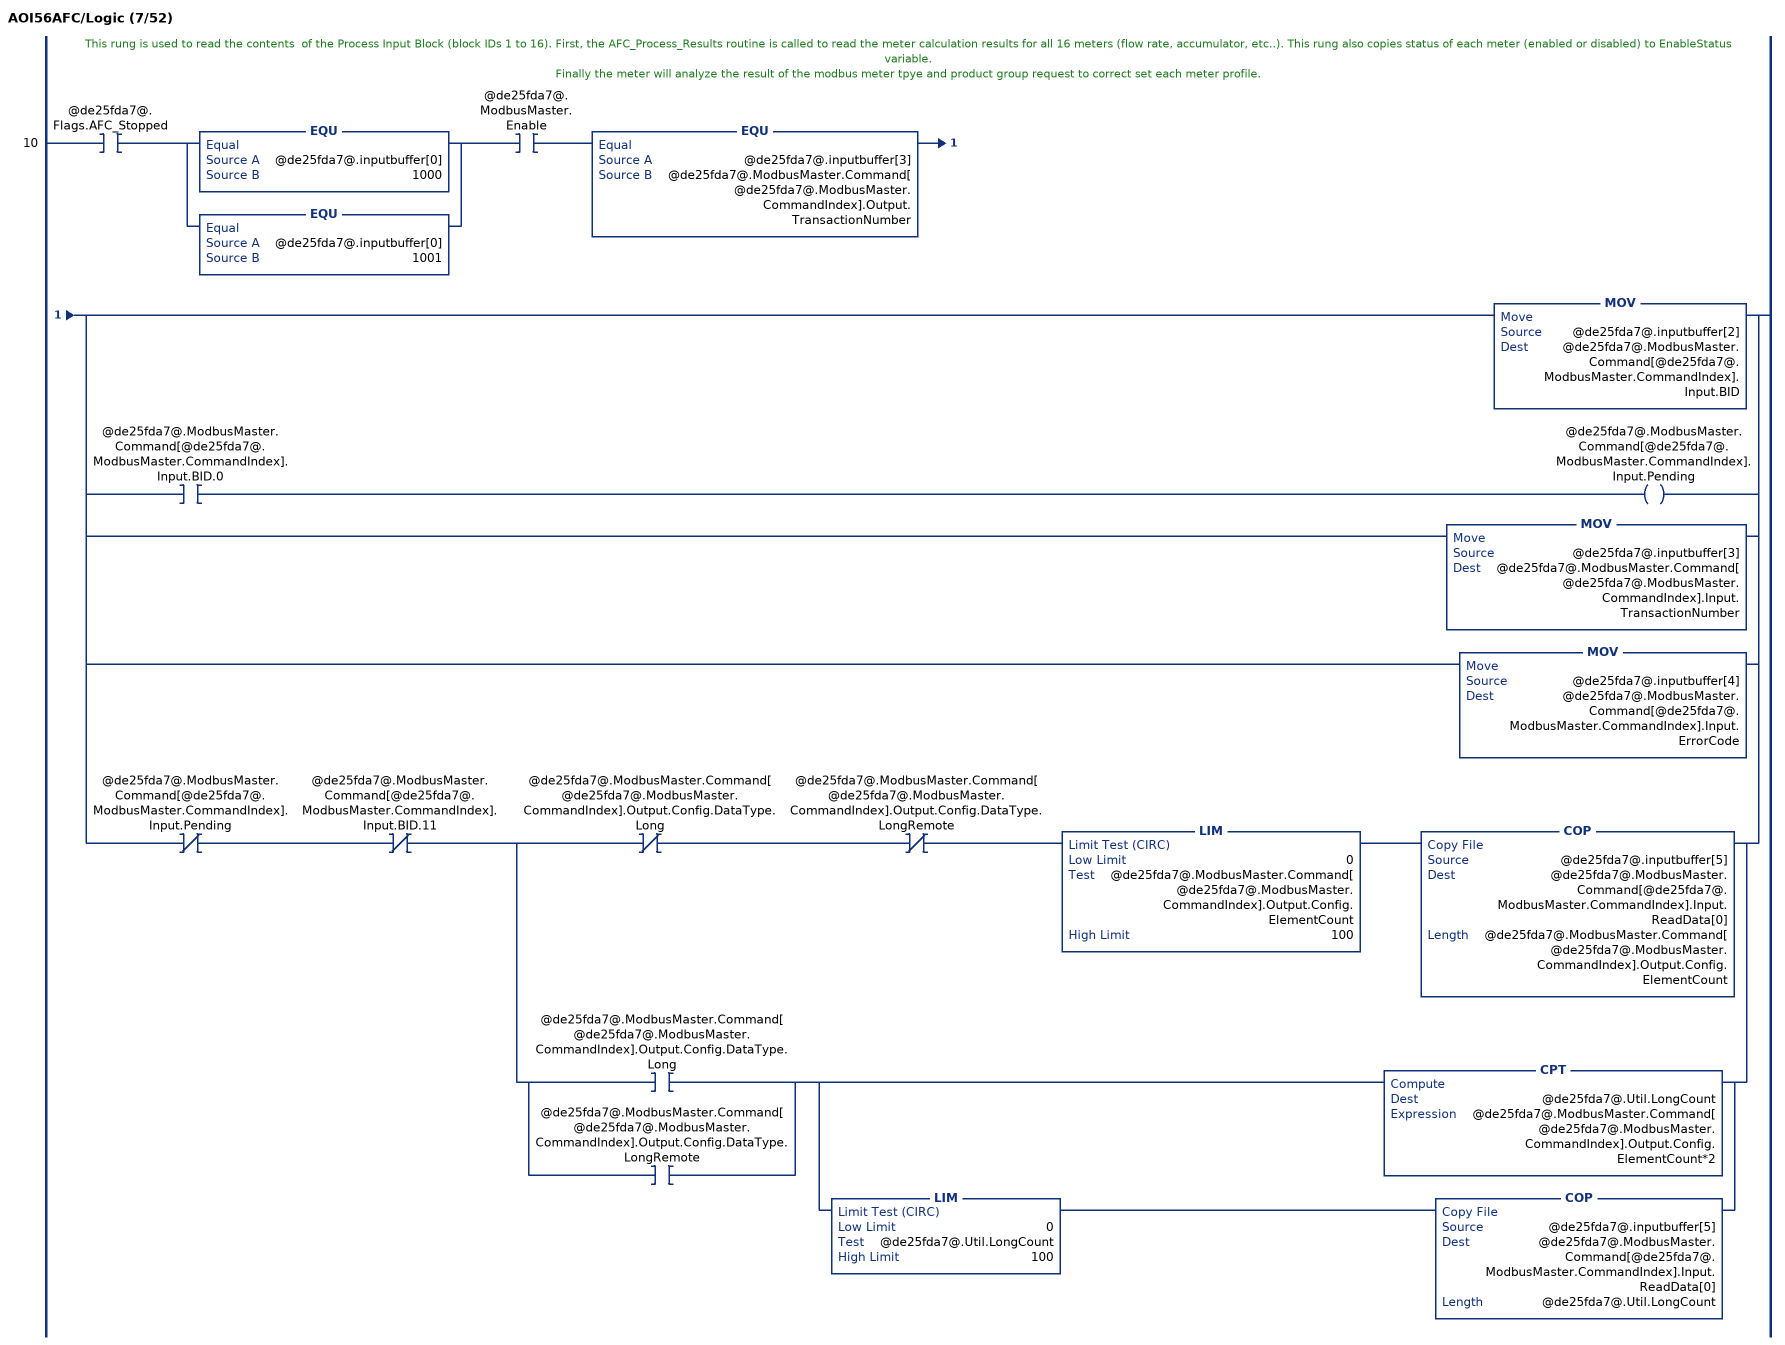
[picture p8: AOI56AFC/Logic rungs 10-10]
   // This rung is used to read the contents  of the Process Input Block (block IDs 1 to 16). First, the AFC_Process_Results routine is called to read the meter calculation results for all 16 meters (flow rate, accumulator, etc..). This rung also copies status of each meter (enabled or disabled) to EnableStatus variable.
   // Finally the meter will analyze the result of the modbus meter tpye and product group request to correct set each meter profile.
   10: XIC(@de25fda7@.Flags.AFC_Stopped)[EQU(@de25fda7@.inputbuffer[0],1000) ,EQU(@de25fda7@.inputbuffer[0],1001) ]XIC(@de25fda7@.ModbusMaster.Enable)EQU(@de25fda7@.inputbuffer[3],@de25fda7@.ModbusMaster.Command[@de25fda7@.ModbusMaster.CommandIndex].Output.TransactionNumber)[MOV(@de25fda7@.inputbuffer[2],@de25fda7@.ModbusMaster.Command[@de25fda7@.ModbusMaster.CommandIndex].Input.BID) ,XIC(@de25fda7@.ModbusMaster.Command[@de25fda7@.ModbusMaster.CommandIndex].Input.BID.0) OTE(@de25fda7@.ModbusMaster.Command[@de25fda7@.ModbusMaster.CommandIndex].Input.Pending) ,MOV(@de25fda7@.inputbuffer[3],@de25fda7@.ModbusMaster.Command[@de25fda7@.ModbusMaster.CommandIndex].Input.TransactionNumber) ,MOV(@de25fda7@.inputbuffer[4],@de25fda7@.ModbusMaster.Command[@de25fda7@.ModbusMaster.CommandIndex].Input.ErrorCode) ,XIO(@de25fda7@.ModbusMaster.Command[@de25fda7@.ModbusMaster.CommandIndex].Input.Pending) XIO(@de25fda7@.ModbusMaster.Command[@de25fda7@.ModbusMaster.CommandIndex].Input.BID.11) [XIO(@de25fda7@.ModbusMaster.Command[@de25fda7@.ModbusMaster.CommandIndex].Output.Config.DataType.Long) XIO(@de25fda7@.ModbusMaster.Command[@de25fda7@.ModbusMaster.CommandIndex].Output.Config.DataType.LongRemote) LIM(0,@de25fda7@.ModbusMaster.Command[@de25fda7@.ModbusMaster.CommandIndex].Output.Config.ElementCount,100) COP(@de25fda7@.inputbuffer[5],@de25fda7@.ModbusMaster.Command[@de25fda7@.ModbusMaster.CommandIndex].Input.ReadData[0],@de25fda7@.ModbusMaster.Command[@de25fda7@.ModbusMaster.CommandIndex].Output.Config.ElementCount) ,[XIC(@de25fda7@.ModbusMaster.Command[@de25fda7@.ModbusMaster.CommandIndex].Output.Config.DataType.Long) ,XIC(@de25fda7@.ModbusMaster.Command[@de25fda7@.ModbusMaster.CommandIndex].Output.Config.DataType.LongRemote) ] [CPT(@de25fda7@.Util.LongCount,@de25fda7@.ModbusMaster.Command[@de25fda7@.ModbusMaster.CommandIndex].Output.Config.ElementCount*2) ,LIM(0,@de25fda7@.Util.LongCount,100) COP(@de25fda7@.inputbuffer[5],@de25fda7@.ModbusMaster.Command[@de25fda7@.ModbusMaster.CommandIndex].Input.ReadData[0],@de25fda7@.Util.LongCount) ] ] ];
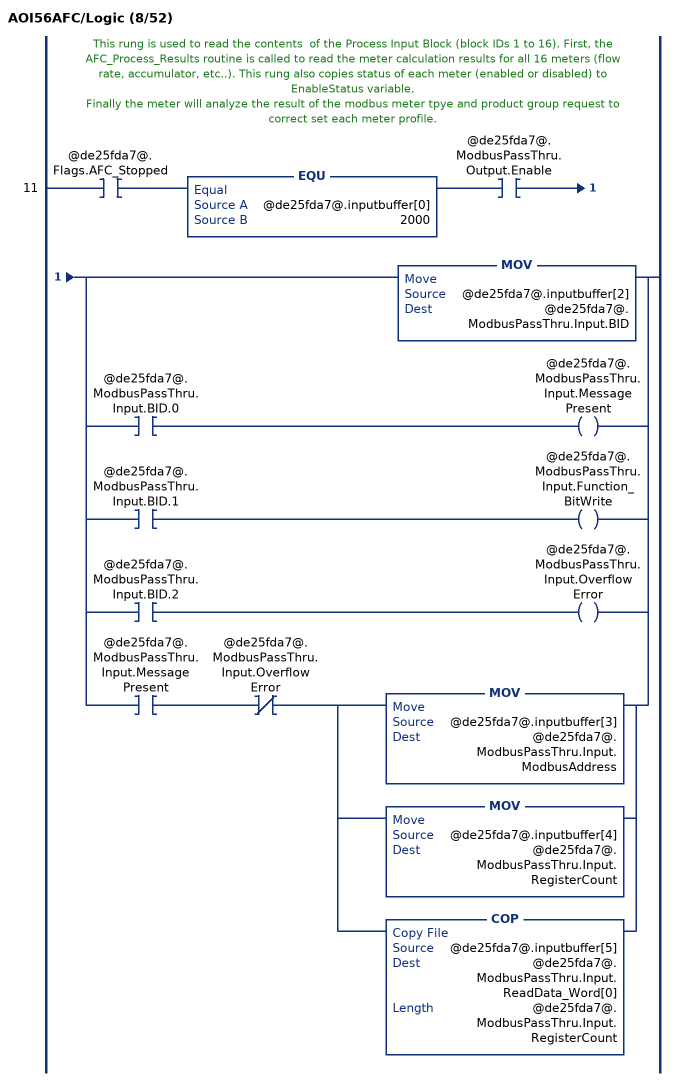
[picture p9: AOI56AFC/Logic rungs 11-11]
   // This rung is used to read the contents  of the Process Input Block (block IDs 1 to 16). First, the AFC_Process_Results routine is called to read the meter calculation results for all 16 meters (flow rate, accumulator, etc..). This rung also copies status of each meter (enabled or disabled) to EnableStatus variable.
   // Finally the meter will analyze the result of the modbus meter tpye and product group request to correct set each meter profile.
   11: XIC(@de25fda7@.Flags.AFC_Stopped)EQU(@de25fda7@.inputbuffer[0],2000)XIC(@de25fda7@.ModbusPassThru.Output.Enable)[MOV(@de25fda7@.inputbuffer[2],@de25fda7@.ModbusPassThru.Input.BID) ,XIC(@de25fda7@.ModbusPassThru.Input.BID.0) OTE(@de25fda7@.ModbusPassThru.Input.MessagePresent) ,XIC(@de25fda7@.ModbusPassThru.Input.BID.1) OTE(@de25fda7@.ModbusPassThru.Input.Function_BitWrite) ,XIC(@de25fda7@.ModbusPassThru.Input.BID.2) OTE(@de25fda7@.ModbusPassThru.Input.OverflowError) ,XIC(@de25fda7@.ModbusPassThru.Input.MessagePresent) XIO(@de25fda7@.ModbusPassThru.Input.OverflowError) [MOV(@de25fda7@.inputbuffer[3],@de25fda7@.ModbusPassThru.Input.ModbusAddress) ,MOV(@de25fda7@.inputbuffer[4],@de25fda7@.ModbusPassThru.Input.RegisterCount) ,COP(@de25fda7@.inputbuffer[5],@de25fda7@.ModbusPassThru.Input.ReadData_Word[0],@de25fda7@.ModbusPassThru.Input.RegisterCount) ] ];
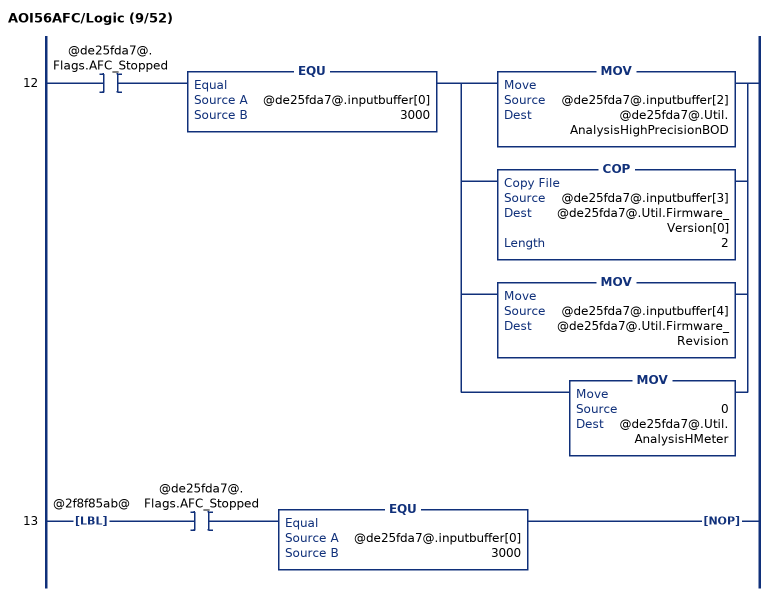
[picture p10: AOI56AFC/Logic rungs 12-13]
   12: XIC(@de25fda7@.Flags.AFC_Stopped)EQU(@de25fda7@.inputbuffer[0],3000)[MOV(@de25fda7@.inputbuffer[2],@de25fda7@.Util.AnalysisHighPrecisionBOD) ,COP(@de25fda7@.inputbuffer[3],@de25fda7@.Util.Firmware_Version[0],2) ,MOV(@de25fda7@.inputbuffer[4],@de25fda7@.Util.Firmware_Revision) ,MOV(0,@de25fda7@.Util.AnalysisHMeter) ];
   13: LBL(@2f8f85ab@)XIC(@de25fda7@.Flags.AFC_Stopped)EQU(@de25fda7@.inputbuffer[0],3000)NOP();
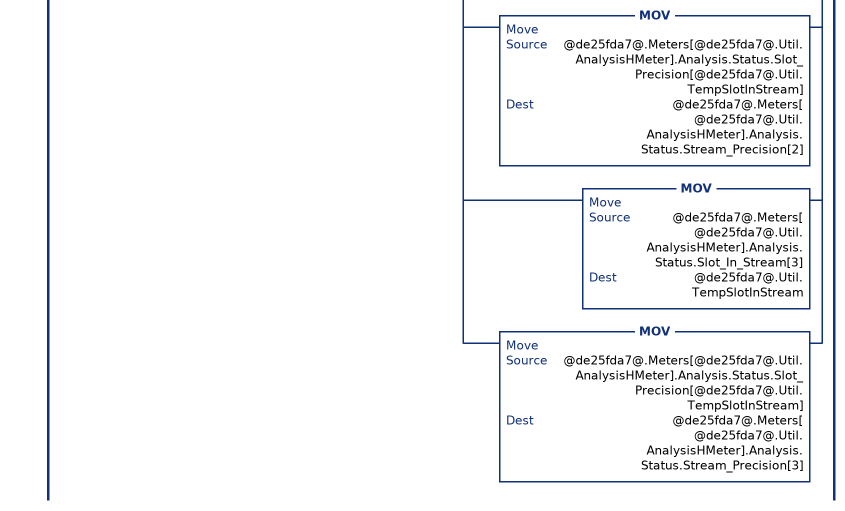
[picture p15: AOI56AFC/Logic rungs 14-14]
   14: XIC(@de25fda7@.Flags.AFC_Stopped)EQU(@de25fda7@.inputbuffer[0],3000)[MOV(0,@de25fda7@.Util.SlotPrecision[0]) ,MOV(0,@de25fda7@.Util.SlotPrecision[1]) ,MOV(0,@de25fda7@.Util.SlotPrecision[2]) ,MOV(0,@de25fda7@.Util.SlotPrecision[3]) ,MVM(@de25fda7@.inputbuffer[5+@de25fda7@.Util.AnalysisHMeter],3,@de25fda7@.Util.SlotPrecision[0]) ,MOV(@de25fda7@.Util.SlotPrecision[0],@de25fda7@.Meters[@de25fda7@.Util.AnalysisHMeter].Analysis.Status.Slot_Precision[0]) ,MVM(@de25fda7@.inputbuffer[5+@de25fda7@.Util.AnalysisHMeter],12,@de25fda7@.Util.SlotPrecision[1]) ,DIV(@de25fda7@.Util.SlotPrecision[1],4,@de25fda7@.Meters[@de25fda7@.Util.AnalysisHMeter].Analysis.Status.Slot_Precision[1]) ,MVM(@de25fda7@.inputbuffer[5+@de25fda7@.Util.AnalysisHMeter],48,@de25fda7@.Util.SlotPrecision[2]) ,DIV(@de25fda7@.Util.SlotPrecision[2],16,@de25fda7@.Meters[@de25fda7@.Util.AnalysisHMeter].Analysis.Status.Slot_Precision[2]) ,MVM(@de25fda7@.inputbuffer[5+@de25fda7@.Util.AnalysisHMeter],192,@de25fda7@.Util.SlotPrecision[3]) ,DIV(@de25fda7@.Util.SlotPrecision[3],64,@de25fda7@.Meters[@de25fda7@.Util.AnalysisHMeter].Analysis.Status.Slot_Precision[3]) ,MOV(0,@de25fda7@.Util.SlotInStream[0]) ,MOV(0,@de25fda7@.Util.SlotInStream[1]) ,MOV(0,@de25fda7@.Util.SlotInStream[2]) ,MOV(0,@de25fda7@.Util.SlotInStream[3]) ,MVM(@de25fda7@.inputbuffer[5+@de25fda7@.Util.AnalysisHMeter],768,@de25fda7@.Util.SlotInStream[0]) ,DIV(@de25fda7@.Util.SlotInStream[0],256,@de25fda7@.Meters[@de25fda7@.Util.AnalysisHMeter].Analysis.Status.Slot_In_Stream[0]) ,MVM(@de25fda7@.inputbuffer[5+@de25fda7@.Util.AnalysisHMeter],3072,@de25fda7@.Util.SlotInStream[1]) ,DIV(@de25fda7@.Util.SlotInStream[1],1024,@de25fda7@.Meters[@de25fda7@.Util.AnalysisHMeter].Analysis.Status.Slot_In_Stream[1]) ,MVM(@de25fda7@.inputbuffer[5+@de25fda7@.Util.AnalysisHMeter],12288,@de25fda7@.Util.SlotInStream[2]) ,DIV(@de25fda7@.Util.SlotInStream[2],4096,@de25fda7@.Meters[@de25fda7@.Util.AnalysisHMeter].Analysis.Status.Slot_In_Stream[2]) ,MVM(@de25fda7@.inputbuffer[5+@de25fda7@.Util.AnalysisHMeter],49152,@de25fda7@.Util.SlotInStream[3]) ,DIV(@de25fda7@.Util.SlotInStream[3],16384,@de25fda7@.Meters[@de25fda7@.Util.AnalysisHMeter].Analysis.Status.Slot_In_Stream[3]) ,MOV(@de25fda7@.Meters[@de25fda7@.Util.AnalysisHMeter].Analysis.Status.Slot_In_Stream[0],@de25fda7@.Util.TempSlotInStream) ,MOV(@de25fda7@.Meters[@de25fda7@.Util.AnalysisHMeter].Analysis.Status.Slot_Precision[@de25fda7@.Util.TempSlotInStream],@de25fda7@.Meters[@de25fda7@.Util.AnalysisHMeter].Analysis.Status.Stream_Precision[0]) ,MOV(@de25fda7@.Meters[@de25fda7@.Util.AnalysisHMeter].Analysis.Status.Slot_In_Stream[1],@de25fda7@.Util.TempSlotInStream) ,MOV(@de25fda7@.Meters[@de25fda7@.Util.AnalysisHMeter].Analysis.Status.Slot_Precision[@de25fda7@.Util.TempSlotInStream],@de25fda7@.Meters[@de25fda7@.Util.AnalysisHMeter].Analysis.Status.Stream_Precision[1]) ,MOV(@de25fda7@.Meters[@de25fda7@.Util.AnalysisHMeter].Analysis.Status.Slot_In_Stream[2],@de25fda7@.Util.TempSlotInStream) ,MOV(@de25fda7@.Meters[@de25fda7@.Util.AnalysisHMeter].Analysis.Status.Slot_Precision[@de25fda7@.Util.TempSlotInStream],@de25fda7@.Meters[@de25fda7@.Util.AnalysisHMeter].Analysis.Status.Stream_Precision[2]) ,MOV(@de25fda7@.Meters[@de25fda7@.Util.AnalysisHMeter].Analysis.Status.Slot_In_Stream[3],@de25fda7@.Util.TempSlotInStream) ,MOV(@de25fda7@.Meters[@de25fda7@.Util.AnalysisHMeter].Analysis.Status.Slot_Precision[@de25fda7@.Util.TempSlotInStream],@de25fda7@.Meters[@de25fda7@.Util.AnalysisHMeter].Analysis.Status.Stream_Precision[3]) ];
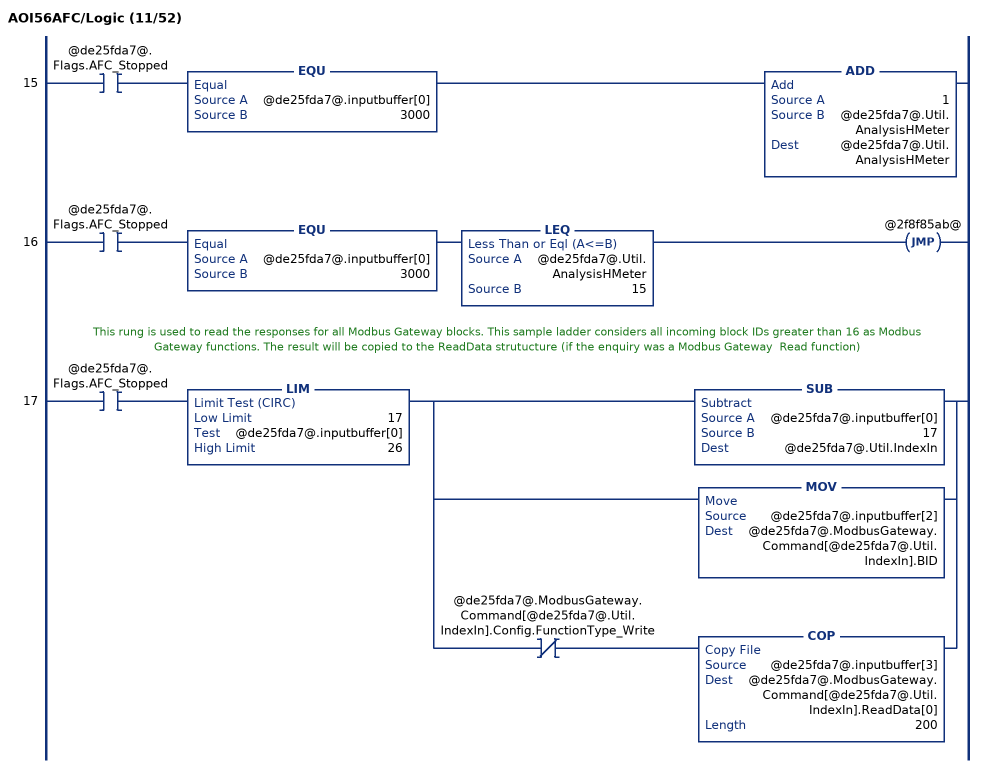
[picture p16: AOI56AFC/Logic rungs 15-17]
   15: XIC(@de25fda7@.Flags.AFC_Stopped)EQU(@de25fda7@.inputbuffer[0],3000)ADD(1,@de25fda7@.Util.AnalysisHMeter,@de25fda7@.Util.AnalysisHMeter);
   16: XIC(@de25fda7@.Flags.AFC_Stopped)EQU(@de25fda7@.inputbuffer[0],3000)LEQ(@de25fda7@.Util.AnalysisHMeter,15)JMP(@2f8f85ab@);
   // This rung is used to read the responses for all Modbus Gateway blocks. This sample ladder considers all incoming block IDs greater than 16 as Modbus Gateway functions. The result will be copied to the ReadData strutucture (if the enquiry was a Modbus Gateway  Read function)
   17: XIC(@de25fda7@.Flags.AFC_Stopped)LIM(17,@de25fda7@.inputbuffer[0],26)[SUB(@de25fda7@.inputbuffer[0],17,@de25fda7@.Util.IndexIn) ,MOV(@de25fda7@.inputbuffer[2],@de25fda7@.ModbusGateway.Command[@de25fda7@.Util.IndexIn].BID) ,XIO(@de25fda7@.ModbusGateway.Command[@de25fda7@.Util.IndexIn].Config.FunctionType_Write) COP(@de25fda7@.inputbuffer[3],@de25fda7@.ModbusGateway.Command[@de25fda7@.Util.IndexIn].ReadData[0],200) ];
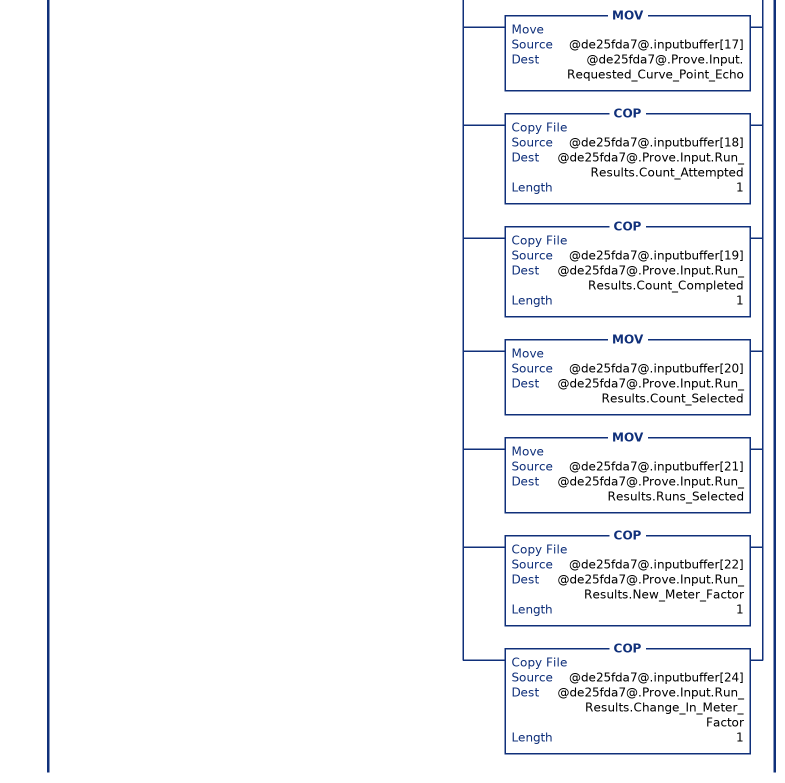
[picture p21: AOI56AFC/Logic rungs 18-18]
   18: XIC(@de25fda7@.Flags.AFC_Stopped)EQU(@de25fda7@.inputbuffer[0],5000)[XIC(@de25fda7@.Util.Prover_Signals.1) OTU(@de25fda7@.Prove.Output.Signals.EnableProve) ,XIC(@de25fda7@.Util.Prover_Signals.2) OTU(@de25fda7@.Prove.Output.Signals.AcceptProve) ,XIC(@de25fda7@.Util.Prover_Signals.3) OTU(@de25fda7@.Prove.Output.Signals.RejectProve) ,XIC(@de25fda7@.Util.Prover_Signals.4) OTU(@de25fda7@.Prove.Output.Signals.RunStart) ,XIC(@de25fda7@.Util.Prover_Signals.5) OTU(@de25fda7@.Prove.Output.Signals.RunComplete) ,XIC(@de25fda7@.Util.Prover_Signals.6) OTU(@de25fda7@.Prove.Output.Signals.RunCancel) ,XIC(@de25fda7@.Util.Prover_Signals.7) OTU(@de25fda7@.Prove.Output.Signals.RunDelete) ,XIC(@de25fda7@.Util.Prover_Signals.9) OTU(@de25fda7@.Prove.Output.Signals.PassComplete) ,XIC(@de25fda7@.Util.Prover_Signals.12) OTU(@de25fda7@.Prove.Output.Signals.PauseProve) ,XIC(@de25fda7@.Util.Prover_Signals.14) OTU(@de25fda7@.Prove.Output.Signals.AbortProve) ,MOV(@de25fda7@.inputbuffer[3],@de25fda7@.Prove.Input.Config.Type) ,MOV(@de25fda7@.inputbuffer[4],@de25fda7@.Prove.Input.Config.Options) ,MOV(@de25fda7@.inputbuffer[5],@de25fda7@.Prove.Input.Config.Runs_per_prove_total) ,MOV(@de25fda7@.inputbuffer[6],@de25fda7@.Prove.Input.Config.Runs_per_prove_selected) ,MOV(@de25fda7@.inputbuffer[7],@de25fda7@.Prove.Input.Config.Max_Runs_before_Abort) ,MOV(@de25fda7@.inputbuffer[8],@de25fda7@.Prove.Input.Config.Short_passes_per_run) ,XIC(@de25fda7@.inputbuffer[12].0) OTL(@de25fda7@.Prove.Input.Status.Prove_Accepted) ,XIO(@de25fda7@.inputbuffer[12].0) OTU(@de25fda7@.Prove.Input.Status.Prove_Accepted) ,XIC(@de25fda7@.inputbuffer[12].1) OTL(@de25fda7@.Prove.Input.Status.Meter_Factor_Applied) ,XIO(@de25fda7@.inputbuffer[12].1) OTU(@de25fda7@.Prove.Input.Status.Meter_Factor_Applied) ,XIC(@de25fda7@.inputbuffer[12].2) OTL(@de25fda7@.Prove.Input.Status.MF_Applied_To_Curve) ,XIO(@de25fda7@.inputbuffer[12].2) OTU(@de25fda7@.Prove.Input.Status.MF_Applied_To_Curve) ,XIC(@de25fda7@.inputbuffer[12].3) OTL(@de25fda7@.Prove.Input.Status.MF_Applied_To_Streams) ,XIO(@de25fda7@.inputbuffer[12].3) OTU(@de25fda7@.Prove.Input.Status.MF_Applied_To_Streams) ,XIC(@de25fda7@.inputbuffer[12].4) OTL(@de25fda7@.Prove.Input.Status.Prove_Rejected_By_Command) ,XIO(@de25fda7@.inputbuffer[12].4) OTU(@de25fda7@.Prove.Input.Status.Prove_Rejected_By_Command) ,XIC(@de25fda7@.inputbuffer[12].5) OTL(@de25fda7@.Prove.Input.Status.Prove_Rejected_No_Runs) ,XIO(@de25fda7@.inputbuffer[12].5) OTU(@de25fda7@.Prove.Input.Status.Prove_Rejected_No_Runs) ,XIC(@de25fda7@.inputbuffer[12].6) OTL(@de25fda7@.Prove.Input.Status.Prove_Rejected_Divide_By_0) ,XIO(@de25fda7@.inputbuffer[12].6) OTU(@de25fda7@.Prove.Input.Status.Prove_Rejected_Divide_By_0) ,XIC(@de25fda7@.inputbuffer[12].8) OTL(@de25fda7@.Prove.Input.Status.Prove_Enabled) ,[XIO(@de25fda7@.inputbuffer[12].8) ,XIC(@de25fda7@.Util.Prover_Signals.2) ,XIC(@de25fda7@.Util.Prover_Signals.3) ,XIC(@de25fda7@.Util.Prover_Signals.14) ] OTU(@de25fda7@.Prove.Input.Status.Prove_Enabled) ,XIC(@de25fda7@.inputbuffer[12].9) OTL(@de25fda7@.Prove.Input.Status.Proving_Run_In_Progress) ,XIO(@de25fda7@.inputbuffer[12].9) OTU(@de25fda7@.Prove.Input.Status.Proving_Run_In_Progress) ,XIC(@de25fda7@.inputbuffer[12].10) OTL(@de25fda7@.Prove.Input.Status.Prove_Paused) ,XIO(@de25fda7@.inputbuffer[12].10) OTU(@de25fda7@.Prove.Input.Status.Prove_Paused) ,XIC(@de25fda7@.inputbuffer[12].11) OTL(@de25fda7@.Prove.Input.Status.Run_Cancelled) ,XIO(@de25fda7@.inputbuffer[12].11) OTU(@de25fda7@.Prove.Input.Status.Run_Cancelled) ,XIC(@de25fda7@.inputbuffer[12].12) OTL(@de25fda7@.Prove.Input.Status.Run_Timed_Out) ,XIO(@de25fda7@.inputbuffer[12].12) OTU(@de25fda7@.Prove.Input.Status.Run_Timed_Out) ,XIC(@de25fda7@.inputbuffer[12].14) OTL(@de25fda7@.Prove.Input.Status.Prove_Rejected_Abort) ,XIO(@de25fda7@.inputbuffer[12].14) OTU(@de25fda7@.Prove.Input.Status.Prove_Rejected_Abort) ,MOV(@de25fda7@.inputbuffer[13],@de25fda7@.Prove.Input.Error_Code) ,MOV(@de25fda7@.inputbuffer[14],@de25fda7@.Prove.Input.Prove_controls_echo) ,MOV(@de25fda7@.inputbuffer[15],@de25fda7@.Prove.Input.Requested_Meter_Echo) ,MOV(@de25fda7@.inputbuffer[17],@de25fda7@.Prove.Input.Requested_Curve_Point_Echo) ,COP(@de25fda7@.inputbuffer[18],@de25fda7@.Prove.Input.Run_Results.Count_Attempted,1) ,COP(@de25fda7@.inputbuffer[19],@de25fda7@.Prove.Input.Run_Results.Count_Completed,1) ,MOV(@de25fda7@.inputbuffer[20],@de25fda7@.Prove.Input.Run_Results.Count_Selected) ,MOV(@de25fda7@.inputbuffer[21],@de25fda7@.Prove.Input.Run_Results.Runs_Selected) ,COP(@de25fda7@.inputbuffer[22],@de25fda7@.Prove.Input.Run_Results.New_Meter_Factor,1) ,COP(@de25fda7@.inputbuffer[24],@de25fda7@.Prove.Input.Run_Results.Change_In_Meter_Factor,1) ];
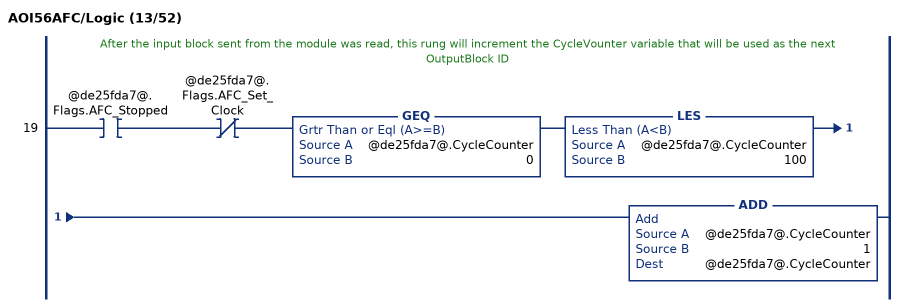
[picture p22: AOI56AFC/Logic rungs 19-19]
   // After the input block sent from the module was read, this rung will increment the CycleVounter variable that will be used as the next OutputBlock ID
   19: XIC(@de25fda7@.Flags.AFC_Stopped)XIO(@de25fda7@.Flags.AFC_Set_Clock)GEQ(@de25fda7@.CycleCounter,0)LES(@de25fda7@.CycleCounter,100)ADD(@de25fda7@.CycleCounter,1,@de25fda7@.CycleCounter);
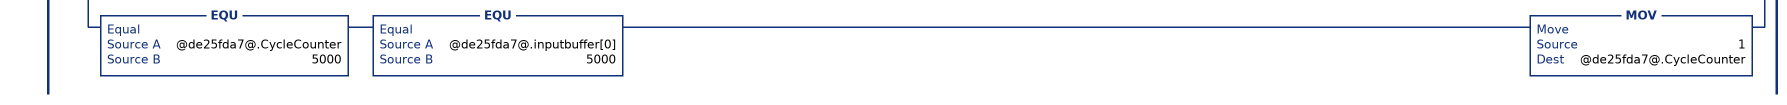
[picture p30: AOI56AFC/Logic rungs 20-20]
   // After the input block sent from the module was read, this rung will increment the CycleVounter variable that will be used as the next OutputBlock ID
   20: XIC(@de25fda7@.Flags.AFC_Stopped)[SUB(@de25fda7@.Util.CycleCounterRollover,1,@de25fda7@.Util.LastRegularBlockID) ,EQU(@de25fda7@.CycleCounter,@de25fda7@.Util.CycleCounterRollover) EQU(@de25fda7@.inputbuffer[0],@de25fda7@.Util.LastRegularBlockID) [XIO(@de25fda7@.ModbusMaster.Enable) XIO(@de25fda7@.ModbusPassThru.Output.Enable) [XIO(@de25fda7@.Prove.Input.Prove_Enabled) MOV(1,@de25fda7@.CycleCounter) ,XIC(@de25fda7@.Prove.Input.Prove_Enabled) MOV(5000,@de25fda7@.CycleCounter) ] ,XIC(@de25fda7@.ModbusMaster.Enable) [MOV(1000,@de25fda7@.CycleCounter) ,OTU(@de25fda7@.ModbusMaster.Command[@de25fda7@.ModbusMaster.CommandIndex].Output.Config.Enable) ] ,XIO(@de25fda7@.ModbusMaster.Enable) XIC(@de25fda7@.ModbusPassThru.Output.Enable) MOV(2000,@de25fda7@.CycleCounter) ,XIO(@de25fda7@.ModbusMaster.Enable) XIO(@de25fda7@.ModbusPassThru.Output.Enable) [XIC(@de25fda7@.Meters[0].Analysis.Status.Update) ,XIC(@de25fda7@.Meters[1].Analysis.Status.Update) ,XIC(@de25fda7@.Meters[2].Analysis.Status.Update) ,XIC(@de25fda7@.Meters[3].Analysis.Status.Update) ,XIC(@de25fda7@.Meters[4].Analysis.Status.Update) ,XIC(@de25fda7@.Meters[5].Analysis.Status.Update) ,XIC(@de25fda7@.Meters[6].Analysis.Status.Update) ,XIC(@de25fda7@.Meters[7].Analysis.Status.Update) ,XIC(@de25fda7@.Meters[8].Analysis.Status.Update) ,XIC(@de25fda7@.Meters[9].Analysis.Status.Update) ,XIC(@de25fda7@.Meters[10].Analysis.Status.Update) ,XIC(@de25fda7@.Meters[11].Analysis.Status.Update) ,XIC(@de25fda7@.Meters[12].Analysis.Status.Update) ,XIC(@de25fda7@.Meters[13].Analysis.Status.Update) ,XIC(@de25fda7@.Meters[14].Analysis.Status.Update) ,XIC(@de25fda7@.Meters[15].Analysis.Status.Update) ] XIC(@de25fda7@.inputbuffer[247].11) MOV(3000,@de25fda7@.CycleCounter) ,XIO(@de25fda7@.ModbusMaster.Enable) XIO(@de25fda7@.ModbusPassThru.Output.Enable) [LES(@de25fda7@.CycleCounter,3000) ,GRT(@de25fda7@.CycleCounter,3004) ] [XIC(@de25fda7@.Meters[0].Analysis.High_Precision.EnableOnce) ,XIC(@de25fda7@.Meters[1].Analysis.High_Precision.EnableOnce) ,XIC(@de25fda7@.Meters[2].Analysis.High_Precision.EnableOnce) ,XIC(@de25fda7@.Meters[3].Analysis.High_Precision.EnableOnce) ,XIC(@de25fda7@.Meters[4].Analysis.High_Precision.EnableOnce) ,XIC(@de25fda7@.Meters[5].Analysis.High_Precision.EnableOnce) ,XIC(@de25fda7@.Meters[6].Analysis.High_Precision.EnableOnce) ,XIC(@de25fda7@.Meters[7].Analysis.High_Precision.EnableOnce) ,XIC(@de25fda7@.Meters[8].Analysis.High_Precision.EnableOnce) ,XIC(@de25fda7@.Meters[9].Analysis.High_Precision.EnableOnce) ,XIC(@de25fda7@.Meters[10].Analysis.High_Precision.EnableOnce) ,XIC(@de25fda7@.Meters[11].Analysis.High_Precision.EnableOnce) ,XIC(@de25fda7@.Meters[12].Analysis.High_Precision.EnableOnce) ,XIC(@de25fda7@.Meters[13].Analysis.High_Precision.EnableOnce) ,XIC(@de25fda7@.Meters[13].Analysis.High_Precision.EnableOnce) ,XIC(@de25fda7@.Meters[14].Analysis.High_Precision.EnableOnce) ,XIC(@de25fda7@.Meters[15].Analysis.High_Precision.EnableOnce) ] XIC(@de25fda7@.inputbuffer[247].11) MOV(3001,@de25fda7@.CycleCounter) ] ,EQU(@de25fda7@.CycleCounter,1000) EQU(@de25fda7@.inputbuffer[0],1000) [MOV(1001,@de25fda7@.CycleCounter) ,OTL(@de25fda7@.ModbusMaster.Command[@de25fda7@.ModbusMaster.CommandIndex].Output.Config.Enable) ] ,EQU(@de25fda7@.CycleCounter,1001) EQU(@de25fda7@.inputbuffer[0],1001) [XIC(@de25fda7@.ModbusPassThru.Output.Enable) MOV(2000,@de25fda7@.CycleCounter) ,XIO(@de25fda7@.ModbusPassThru.Output.Enable) MOV(1,@de25fda7@.CycleCounter) ] ,EQU(@de25fda7@.CycleCounter,2000) EQU(@de25fda7@.inputbuffer[0],2000) MOV(1,@de25fda7@.CycleCounter) ,EQU(@de25fda7@.CycleCounter,3001) EQU(@de25fda7@.inputbuffer[0],3001) MOV(3002,@de25fda7@.CycleCounter) ,EQU(@de25fda7@.CycleCounter,3002) EQU(@de25fda7@.inputbuffer[0],3002) MOV(3003,@de25fda7@.CycleCounter) ,EQU(@de25fda7@.CycleCounter,3003) EQU(@de25fda7@.inputbuffer[0],3003) MOV(3004,@de25fda7@.CycleCounter) ,EQU(@de25fda7@.CycleCounter,3004) EQU(@de25fda7@.inputbuffer[0],3004) [XIO(@de25fda7@.Prove.Input.Prove_Enabled) MOV(1,@de25fda7@.CycleCounter) ,XIC(@de25fda7@.Prove.Input.Prove_Enabled) MOV(5000,@de25fda7@.CycleCounter) ,OTU(@de25fda7@.Meters[0].Analysis.High_Precision.EnableOnce) ,OTU(@de25fda7@.Meters[1].Analysis.High_Precision.EnableOnce) ,OTU(@de25fda7@.Meters[2].Analysis.High_Precision.EnableOnce) ,OTU(@de25fda7@.Meters[3].Analysis.High_Precision.EnableOnce) ,OTU(@de25fda7@.Meters[4].Analysis.High_Precision.EnableOnce) ,OTU(@de25fda7@.Meters[5].Analysis.High_Precision.EnableOnce) ,OTU(@de25fda7@.Meters[6].Analysis.High_Precision.EnableOnce) ,OTU(@de25fda7@.Meters[7].Analysis.High_Precision.EnableOnce) ,OTU(@de25fda7@.Meters[8].Analysis.High_Precision.EnableOnce) ,OTU(@de25fda7@.Meters[9].Analysis.High_Precision.EnableOnce) ,OTU(@de25fda7@.Meters[10].Analysis.High_Precision.EnableOnce) ,OTU(@de25fda7@.Meters[11].Analysis.High_Precision.EnableOnce) ,OTU(@de25fda7@.Meters[12].Analysis.High_Precision.EnableOnce) ,OTU(@de25fda7@.Meters[13].Analysis.High_Precision.EnableOnce) ,OTU(@de25fda7@.Meters[13].Analysis.High_Precision.EnableOnce) ,OTU(@de25fda7@.Meters[14].Analysis.High_Precision.EnableOnce) ,OTU(@de25fda7@.Meters[15].Analysis.High_Precision.EnableOnce) ] ,EQU(@de25fda7@.CycleCounter,3000) EQU(@de25fda7@.inputbuffer[0],3000) [MOV(1,@de25fda7@.CycleCounter) ,OTU(@de25fda7@.Meters[0].Analysis.High_Precision.EnableOnce) ,OTU(@de25fda7@.Meters[1].Analysis.High_Precision.EnableOnce) ,OTU(@de25fda7@.Meters[2].Analysis.High_Precision.EnableOnce) ,OTU(@de25fda7@.Meters[3].Analysis.High_Precision.EnableOnce) ,OTU(@de25fda7@.Meters[4].Analysis.High_Precision.EnableOnce) ,OTU(@de25fda7@.Meters[5].Analysis.High_Precision.EnableOnce) ,OTU(@de25fda7@.Meters[6].Analysis.High_Precision.EnableOnce) ,OTU(@de25fda7@.Meters[7].Analysis.High_Precision.EnableOnce) ,OTU(@de25fda7@.Meters[8].Analysis.High_Precision.EnableOnce) ,OTU(@de25fda7@.Meters[9].Analysis.High_Precision.EnableOnce) ,OTU(@de25fda7@.Meters[10].Analysis.High_Precision.EnableOnce) ,OTU(@de25fda7@.Meters[11].Analysis.High_Precision.EnableOnce) ,OTU(@de25fda7@.Meters[12].Analysis.High_Precision.EnableOnce) ,OTU(@de25fda7@.Meters[13].Analysis.High_Precision.EnableOnce) ,OTU(@de25fda7@.Meters[13].Analysis.High_Precision.EnableOnce) ,OTU(@de25fda7@.Meters[14].Analysis.High_Precision.EnableOnce) ,OTU(@de25fda7@.Meters[15].Analysis.High_Precision.EnableOnce) ] ,[EQU(@de25fda7@.CycleCounter,1000) ,EQU(@de25fda7@.CycleCounter,1001) ] XIO(@de25fda7@.ModbusMaster.Enable) MOV(1,@de25fda7@.CycleCounter) ,EQU(@de25fda7@.CycleCounter,2000) XIO(@de25fda7@.ModbusPassThru.Output.Enable) MOV(1,@de25fda7@.CycleCounter) ,EQU(@de25fda7@.CycleCounter,5000) EQU(@de25fda7@.inputbuffer[0],5000) MOV(1,@de25fda7@.CycleCounter) ];
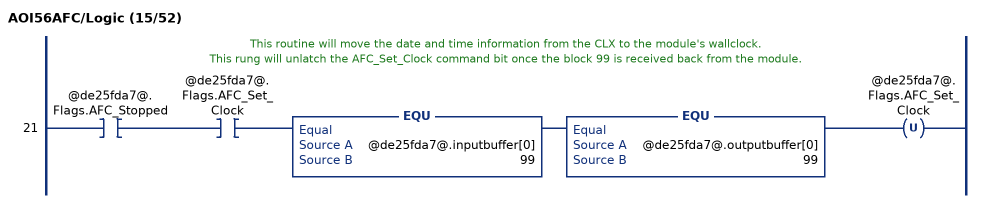
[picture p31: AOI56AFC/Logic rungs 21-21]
   // This routine will move the date and time information from the CLX to the module's wallclock.
   // This rung will unlatch the AFC_Set_Clock command bit once the block 99 is received back from the module.
   21: XIC(@de25fda7@.Flags.AFC_Stopped)XIC(@de25fda7@.Flags.AFC_Set_Clock)EQU(@de25fda7@.inputbuffer[0],99)EQU(@de25fda7@.outputbuffer[0],99)OTU(@de25fda7@.Flags.AFC_Set_Clock);
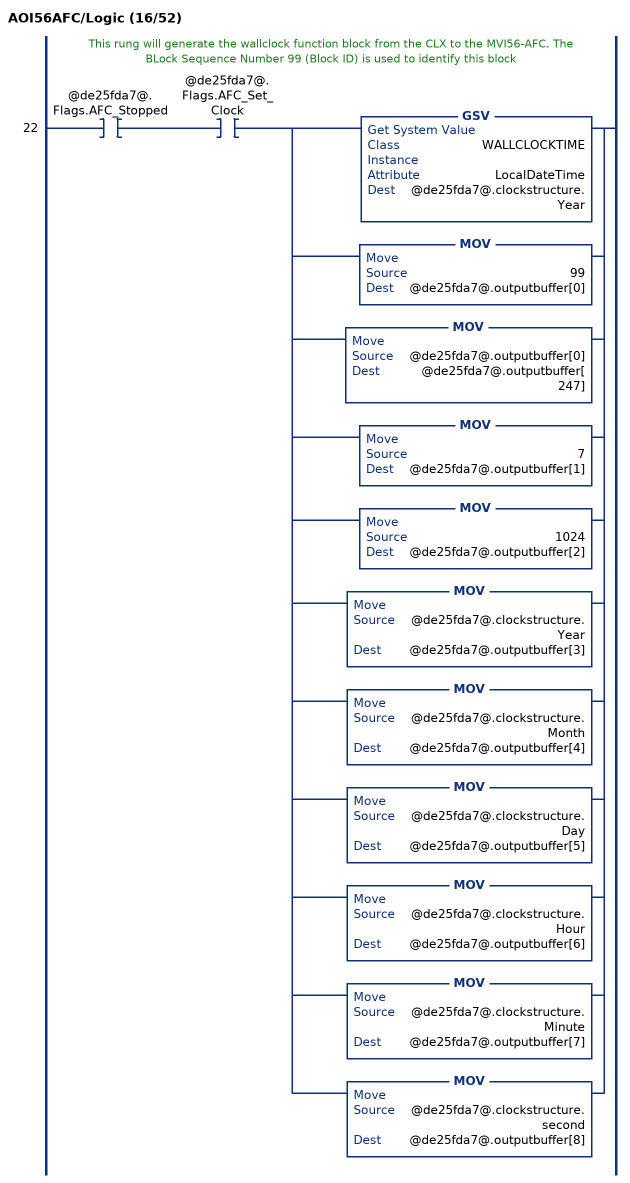
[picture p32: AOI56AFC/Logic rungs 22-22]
   // This rung will generate the wallclock function block from the CLX to the MVI56-AFC. The BLock Sequence Number 99 (Block ID) is used to identify this block
   22: XIC(@de25fda7@.Flags.AFC_Stopped)XIC(@de25fda7@.Flags.AFC_Set_Clock)[GSV(WALLCLOCKTIME,,LocalDateTime,@de25fda7@.clockstructure.Year) ,MOV(99,@de25fda7@.outputbuffer[0]) ,MOV(@de25fda7@.outputbuffer[0],@de25fda7@.outputbuffer[247]) ,MOV(7,@de25fda7@.outputbuffer[1]) ,MOV(1024,@de25fda7@.outputbuffer[2]) ,MOV(@de25fda7@.clockstructure.Year,@de25fda7@.outputbuffer[3]) ,MOV(@de25fda7@.clockstructure.Month,@de25fda7@.outputbuffer[4]) ,MOV(@de25fda7@.clockstructure.Day,@de25fda7@.outputbuffer[5]) ,MOV(@de25fda7@.clockstructure.Hour,@de25fda7@.outputbuffer[6]) ,MOV(@de25fda7@.clockstructure.Minute,@de25fda7@.outputbuffer[7]) ,MOV(@de25fda7@.clockstructure.second,@de25fda7@.outputbuffer[8]) ];
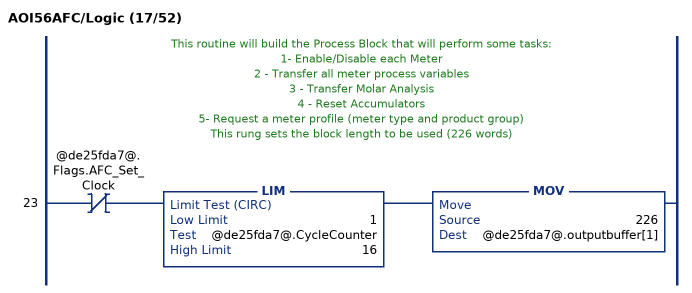
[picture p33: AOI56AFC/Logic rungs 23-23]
   // This routine will build the Process Block that will perform some tasks:
   // 1- Enable/Disable each Meter
   // 2 - Transfer all meter process variables
   // 3 - Transfer Molar Analysis
   // 4 - Reset Accumulators
   // 5- Request a meter profile (meter type and product group)
   // This rung sets the block length to be used (226 words)
   23: XIO(@de25fda7@.Flags.AFC_Set_Clock)LIM(1,@de25fda7@.CycleCounter,16)MOV(226,@de25fda7@.outputbuffer[1]);
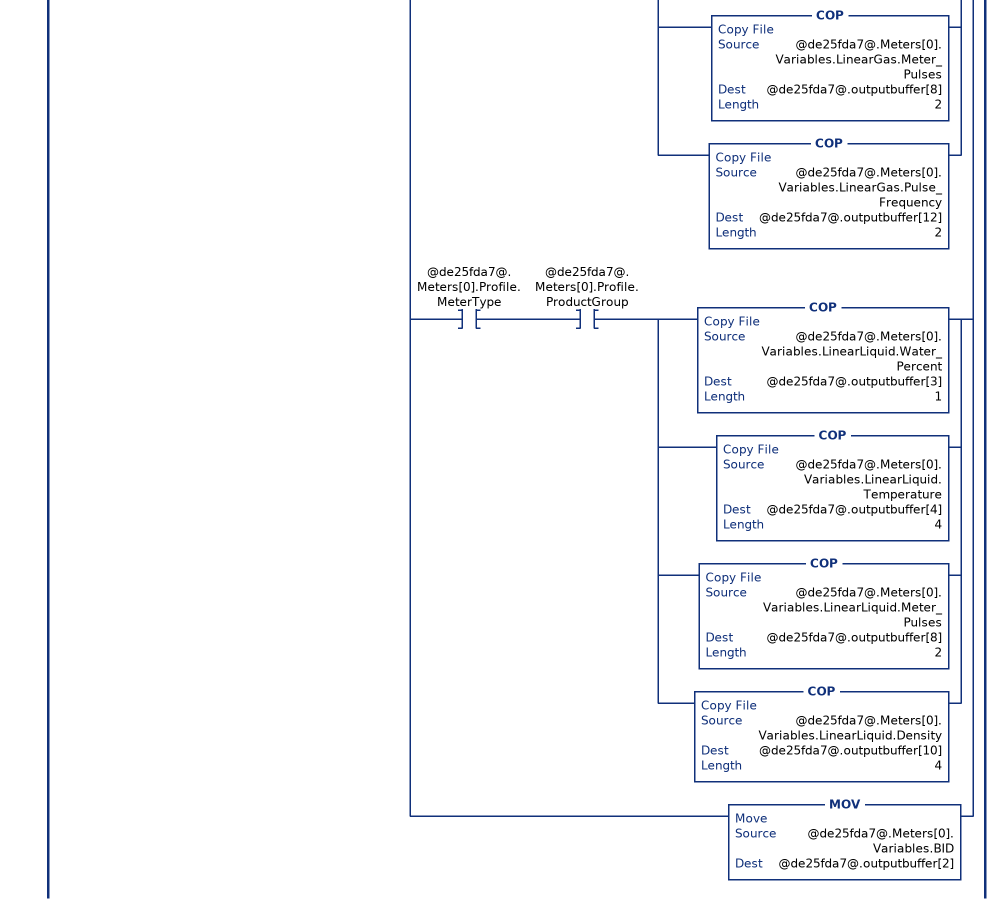
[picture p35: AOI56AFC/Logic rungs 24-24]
   // This routine will copy the meter variables  for all 16 meters from the AFC56.Meters[].Variables data structure to the outputbuffer[] array. The logic will copy the variables according to each meter profile (meter type and product group).
   // This routine also verifies each EnableStatus variable in order to unlatch the meter disable or enable commands.
   24: XIO(@de25fda7@.Flags.AFC_Set_Clock)LIM(1,@de25fda7@.CycleCounter,16)[ADD(1,8192,@de25fda7@.Meters[0].Variables.BID) ,XIO(@de25fda7@.EnableStatus.Meter1) [OTE(@de25fda7@.Meters[0].Variables.BID.8) ,OTU(@de25fda7@.DisableMeter.Meter1) ] ,XIC(@de25fda7@.EnableStatus.Meter1) OTU(@de25fda7@.EnableMeter.Meter1) ,XIO(@de25fda7@.Meters[0].Profile.MeterType) XIO(@de25fda7@.Meters[0].Profile.ProductGroup) COP(@de25fda7@.Meters[0].Variables.DifferentialGas.Temperature,@de25fda7@.outputbuffer[4],6) ,XIO(@de25fda7@.Meters[0].Profile.MeterType) XIC(@de25fda7@.Meters[0].Profile.ProductGroup) [COP(@de25fda7@.Meters[0].Variables.DifferentialLiquid.Water_Percent,@de25fda7@.outputbuffer[3],1) ,COP(@de25fda7@.Meters[0].Variables.DifferentialLiquid.Temperature,@de25fda7@.outputbuffer[4],8) ] ,XIC(@de25fda7@.Meters[0].Profile.MeterType) XIO(@de25fda7@.Meters[0].Profile.ProductGroup) [COP(@de25fda7@.Meters[0].Variables.LinearGas.Temperature,@de25fda7@.outputbuffer[4],4) ,COP(@de25fda7@.Meters[0].Variables.LinearGas.Meter_Pulses,@de25fda7@.outputbuffer[8],2) ,COP(@de25fda7@.Meters[0].Variables.LinearGas.Pulse_Frequency,@de25fda7@.outputbuffer[12],2) ] ,XIC(@de25fda7@.Meters[0].Profile.MeterType) XIC(@de25fda7@.Meters[0].Profile.ProductGroup) [COP(@de25fda7@.Meters[0].Variables.LinearLiquid.Water_Percent,@de25fda7@.outputbuffer[3],1) ,COP(@de25fda7@.Meters[0].Variables.LinearLiquid.Temperature,@de25fda7@.outputbuffer[4],4) ,COP(@de25fda7@.Meters[0].Variables.LinearLiquid.Meter_Pulses,@de25fda7@.outputbuffer[8],2) ,COP(@de25fda7@.Meters[0].Variables.LinearLiquid.Density,@de25fda7@.outputbuffer[10],4) ] ,MOV(@de25fda7@.Meters[0].Variables.BID,@de25fda7@.outputbuffer[2]) ];
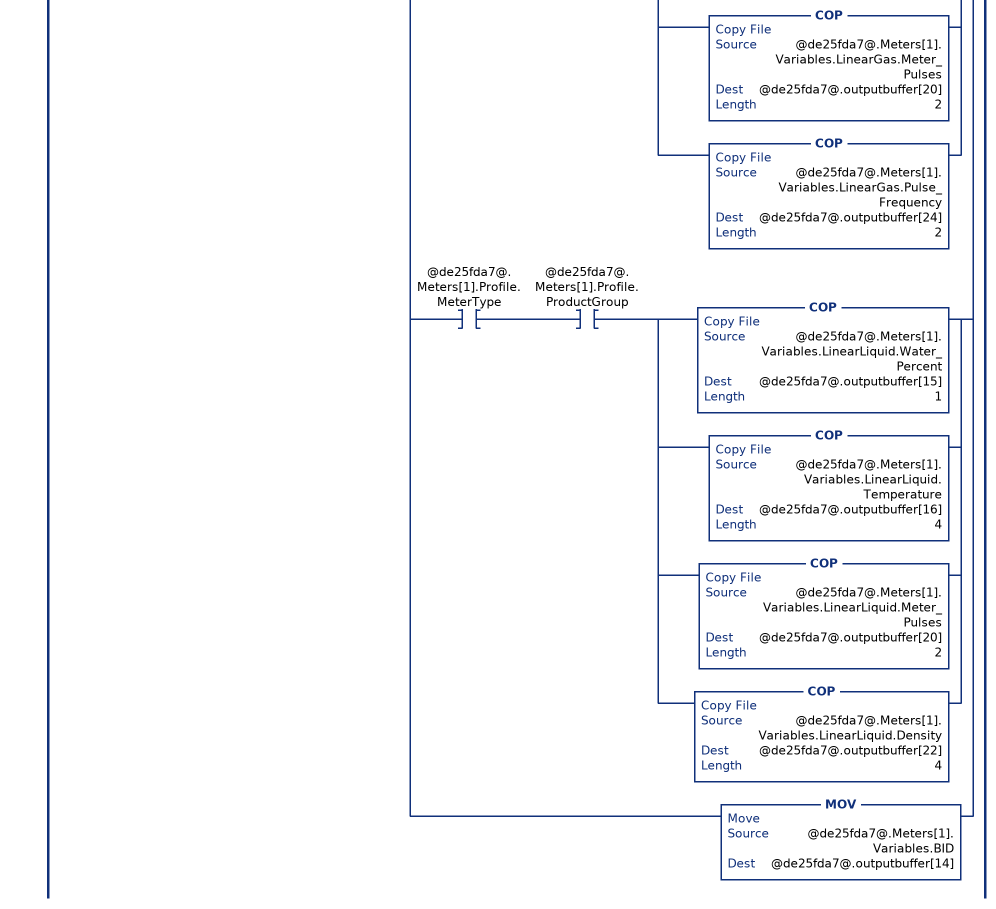
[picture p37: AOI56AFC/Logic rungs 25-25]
   25: XIO(@de25fda7@.Flags.AFC_Set_Clock)LIM(1,@de25fda7@.CycleCounter,16)[ADD(2,8192,@de25fda7@.Meters[1].Variables.BID) ,XIO(@de25fda7@.EnableStatus.Meter2) [OTE(@de25fda7@.Meters[1].Variables.BID.8) ,OTU(@de25fda7@.DisableMeter.Meter2) ] ,XIC(@de25fda7@.EnableStatus.Meter2) OTU(@de25fda7@.EnableMeter.Meter2) ,XIO(@de25fda7@.Meters[1].Profile.MeterType) XIO(@de25fda7@.Meters[1].Profile.ProductGroup) COP(@de25fda7@.Meters[1].Variables.DifferentialGas.Temperature,@de25fda7@.outputbuffer[16],6) ,XIO(@de25fda7@.Meters[1].Profile.MeterType) XIC(@de25fda7@.Meters[1].Profile.ProductGroup) [COP(@de25fda7@.Meters[1].Variables.DifferentialLiquid.Water_Percent,@de25fda7@.outputbuffer[15],1) ,COP(@de25fda7@.Meters[1].Variables.DifferentialLiquid.Temperature,@de25fda7@.outputbuffer[16],8) ] ,XIC(@de25fda7@.Meters[1].Profile.MeterType) XIO(@de25fda7@.Meters[1].Profile.ProductGroup) [COP(@de25fda7@.Meters[1].Variables.LinearGas.Temperature,@de25fda7@.outputbuffer[16],4) ,COP(@de25fda7@.Meters[1].Variables.LinearGas.Meter_Pulses,@de25fda7@.outputbuffer[20],2) ,COP(@de25fda7@.Meters[1].Variables.LinearGas.Pulse_Frequency,@de25fda7@.outputbuffer[24],2) ] ,XIC(@de25fda7@.Meters[1].Profile.MeterType) XIC(@de25fda7@.Meters[1].Profile.ProductGroup) [COP(@de25fda7@.Meters[1].Variables.LinearLiquid.Water_Percent,@de25fda7@.outputbuffer[15],1) ,COP(@de25fda7@.Meters[1].Variables.LinearLiquid.Temperature,@de25fda7@.outputbuffer[16],4) ,COP(@de25fda7@.Meters[1].Variables.LinearLiquid.Meter_Pulses,@de25fda7@.outputbuffer[20],2) ,COP(@de25fda7@.Meters[1].Variables.LinearLiquid.Density,@de25fda7@.outputbuffer[22],4) ] ,MOV(@de25fda7@.Meters[1].Variables.BID,@de25fda7@.outputbuffer[14]) ];
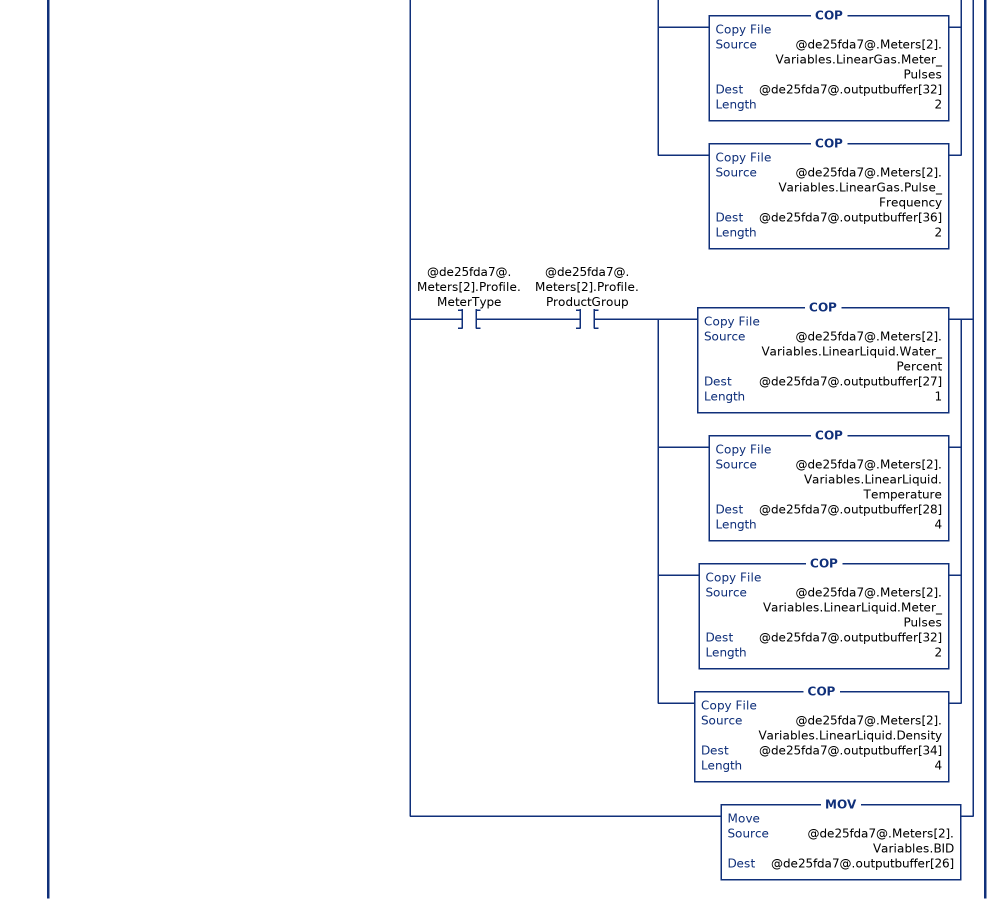
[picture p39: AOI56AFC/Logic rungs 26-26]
   26: XIO(@de25fda7@.Flags.AFC_Set_Clock)LIM(1,@de25fda7@.CycleCounter,16)[ADD(3,8192,@de25fda7@.Meters[2].Variables.BID) ,XIO(@de25fda7@.EnableStatus.Meter3) [OTE(@de25fda7@.Meters[2].Variables.BID.8) ,OTU(@de25fda7@.DisableMeter.Meter3) ] ,XIC(@de25fda7@.EnableStatus.Meter3) OTU(@de25fda7@.EnableMeter.Meter3) ,XIO(@de25fda7@.Meters[2].Profile.MeterType) XIO(@de25fda7@.Meters[2].Profile.ProductGroup) COP(@de25fda7@.Meters[2].Variables.DifferentialGas.Temperature,@de25fda7@.outputbuffer[28],6) ,XIO(@de25fda7@.Meters[2].Profile.MeterType) XIC(@de25fda7@.Meters[2].Profile.ProductGroup) [COP(@de25fda7@.Meters[2].Variables.DifferentialLiquid.Water_Percent,@de25fda7@.outputbuffer[27],1) ,COP(@de25fda7@.Meters[2].Variables.DifferentialLiquid.Temperature,@de25fda7@.outputbuffer[28],8) ] ,XIC(@de25fda7@.Meters[2].Profile.MeterType) XIO(@de25fda7@.Meters[2].Profile.ProductGroup) [COP(@de25fda7@.Meters[2].Variables.LinearGas.Temperature,@de25fda7@.outputbuffer[28],4) ,COP(@de25fda7@.Meters[2].Variables.LinearGas.Meter_Pulses,@de25fda7@.outputbuffer[32],2) ,COP(@de25fda7@.Meters[2].Variables.LinearGas.Pulse_Frequency,@de25fda7@.outputbuffer[36],2) ] ,XIC(@de25fda7@.Meters[2].Profile.MeterType) XIC(@de25fda7@.Meters[2].Profile.ProductGroup) [COP(@de25fda7@.Meters[2].Variables.LinearLiquid.Water_Percent,@de25fda7@.outputbuffer[27],1) ,COP(@de25fda7@.Meters[2].Variables.LinearLiquid.Temperature,@de25fda7@.outputbuffer[28],4) ,COP(@de25fda7@.Meters[2].Variables.LinearLiquid.Meter_Pulses,@de25fda7@.outputbuffer[32],2) ,COP(@de25fda7@.Meters[2].Variables.LinearLiquid.Density,@de25fda7@.outputbuffer[34],4) ] ,MOV(@de25fda7@.Meters[2].Variables.BID,@de25fda7@.outputbuffer[26]) ];
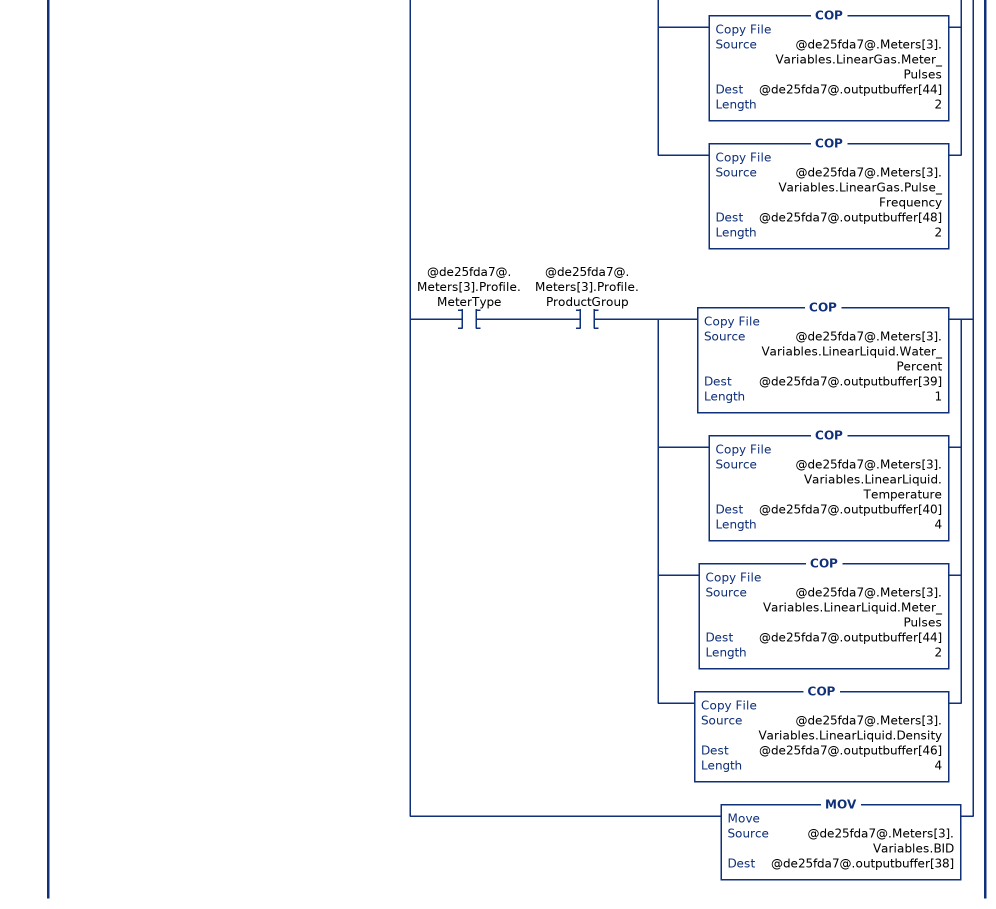
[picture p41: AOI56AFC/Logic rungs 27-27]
   27: XIO(@de25fda7@.Flags.AFC_Set_Clock)LIM(1,@de25fda7@.CycleCounter,16)[ADD(4,8192,@de25fda7@.Meters[3].Variables.BID) ,XIO(@de25fda7@.EnableStatus.Meter4) [OTE(@de25fda7@.Meters[3].Variables.BID.8) ,OTU(@de25fda7@.DisableMeter.Meter4) ] ,XIC(@de25fda7@.EnableStatus.Meter4) OTU(@de25fda7@.EnableMeter.Meter4) ,XIO(@de25fda7@.Meters[3].Profile.MeterType) XIO(@de25fda7@.Meters[3].Profile.ProductGroup) COP(@de25fda7@.Meters[3].Variables.DifferentialGas.Temperature,@de25fda7@.outputbuffer[40],6) ,XIO(@de25fda7@.Meters[3].Profile.MeterType) XIC(@de25fda7@.Meters[3].Profile.ProductGroup) [COP(@de25fda7@.Meters[3].Variables.DifferentialLiquid.Water_Percent,@de25fda7@.outputbuffer[39],1) ,COP(@de25fda7@.Meters[3].Variables.DifferentialLiquid.Temperature,@de25fda7@.outputbuffer[40],8) ] ,XIC(@de25fda7@.Meters[3].Profile.MeterType) XIO(@de25fda7@.Meters[3].Profile.ProductGroup) [COP(@de25fda7@.Meters[3].Variables.LinearGas.Temperature,@de25fda7@.outputbuffer[40],4) ,COP(@de25fda7@.Meters[3].Variables.LinearGas.Meter_Pulses,@de25fda7@.outputbuffer[44],2) ,COP(@de25fda7@.Meters[3].Variables.LinearGas.Pulse_Frequency,@de25fda7@.outputbuffer[48],2) ] ,XIC(@de25fda7@.Meters[3].Profile.MeterType) XIC(@de25fda7@.Meters[3].Profile.ProductGroup) [COP(@de25fda7@.Meters[3].Variables.LinearLiquid.Water_Percent,@de25fda7@.outputbuffer[39],1) ,COP(@de25fda7@.Meters[3].Variables.LinearLiquid.Temperature,@de25fda7@.outputbuffer[40],4) ,COP(@de25fda7@.Meters[3].Variables.LinearLiquid.Meter_Pulses,@de25fda7@.outputbuffer[44],2) ,COP(@de25fda7@.Meters[3].Variables.LinearLiquid.Density,@de25fda7@.outputbuffer[46],4) ] ,MOV(@de25fda7@.Meters[3].Variables.BID,@de25fda7@.outputbuffer[38]) ];
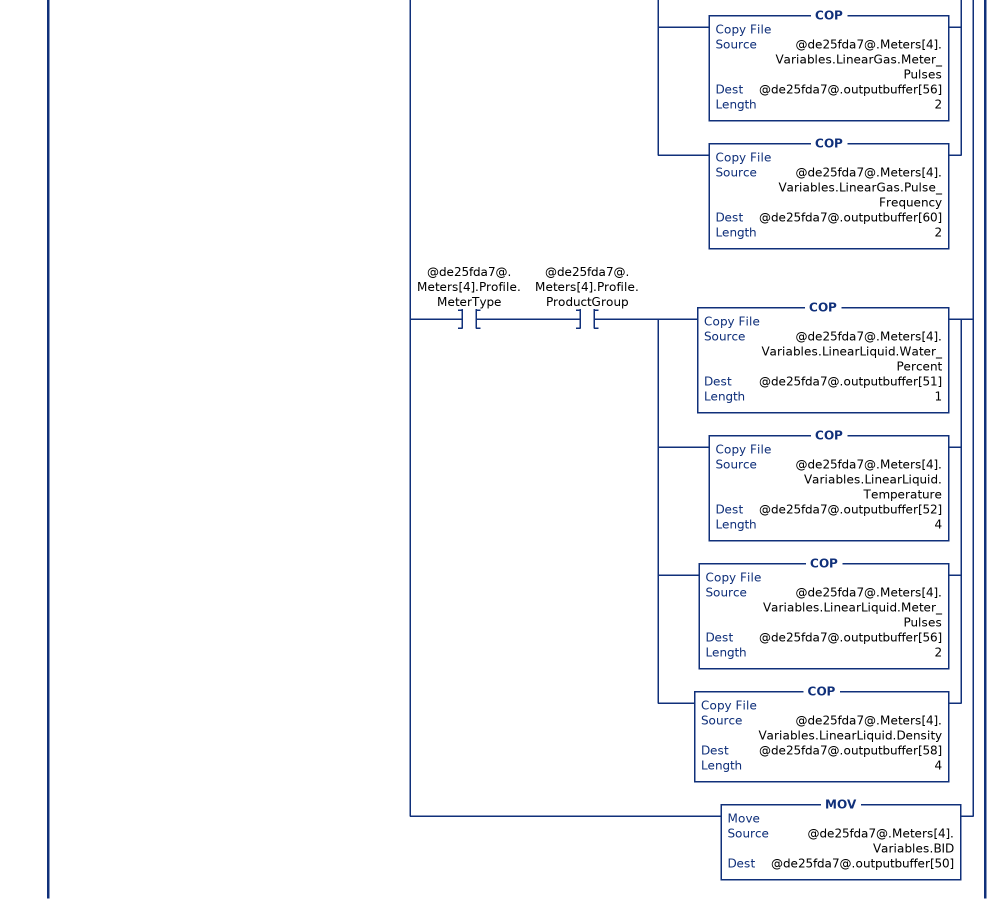
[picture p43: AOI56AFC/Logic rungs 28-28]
   28: XIO(@de25fda7@.Flags.AFC_Set_Clock)LIM(1,@de25fda7@.CycleCounter,16)[ADD(5,8192,@de25fda7@.Meters[4].Variables.BID) ,XIO(@de25fda7@.EnableStatus.Meter5) [OTE(@de25fda7@.Meters[4].Variables.BID.8) ,OTU(@de25fda7@.DisableMeter.Meter5) ] ,XIC(@de25fda7@.EnableStatus.Meter5) OTU(@de25fda7@.EnableMeter.Meter5) ,XIO(@de25fda7@.Meters[4].Profile.MeterType) XIO(@de25fda7@.Meters[4].Profile.ProductGroup) COP(@de25fda7@.Meters[4].Variables.DifferentialGas.Temperature,@de25fda7@.outputbuffer[52],6) ,XIO(@de25fda7@.Meters[4].Profile.MeterType) XIC(@de25fda7@.Meters[4].Profile.ProductGroup) [COP(@de25fda7@.Meters[4].Variables.DifferentialLiquid.Water_Percent,@de25fda7@.outputbuffer[51],1) ,COP(@de25fda7@.Meters[4].Variables.DifferentialLiquid.Temperature,@de25fda7@.outputbuffer[52],8) ] ,XIC(@de25fda7@.Meters[4].Profile.MeterType) XIO(@de25fda7@.Meters[4].Profile.ProductGroup) [COP(@de25fda7@.Meters[4].Variables.LinearGas.Temperature,@de25fda7@.outputbuffer[52],4) ,COP(@de25fda7@.Meters[4].Variables.LinearGas.Meter_Pulses,@de25fda7@.outputbuffer[56],2) ,COP(@de25fda7@.Meters[4].Variables.LinearGas.Pulse_Frequency,@de25fda7@.outputbuffer[60],2) ] ,XIC(@de25fda7@.Meters[4].Profile.MeterType) XIC(@de25fda7@.Meters[4].Profile.ProductGroup) [COP(@de25fda7@.Meters[4].Variables.LinearLiquid.Water_Percent,@de25fda7@.outputbuffer[51],1) ,COP(@de25fda7@.Meters[4].Variables.LinearLiquid.Temperature,@de25fda7@.outputbuffer[52],4) ,COP(@de25fda7@.Meters[4].Variables.LinearLiquid.Meter_Pulses,@de25fda7@.outputbuffer[56],2) ,COP(@de25fda7@.Meters[4].Variables.LinearLiquid.Density,@de25fda7@.outputbuffer[58],4) ] ,MOV(@de25fda7@.Meters[4].Variables.BID,@de25fda7@.outputbuffer[50]) ];
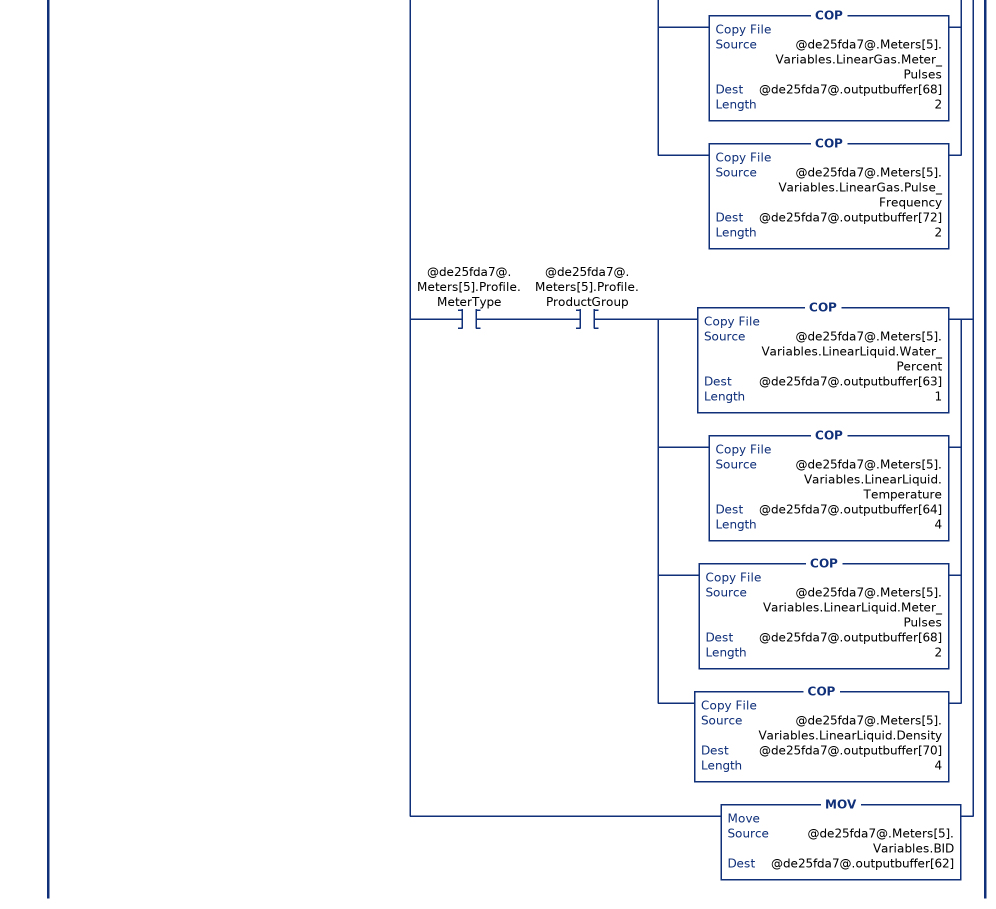
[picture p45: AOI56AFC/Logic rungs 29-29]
   29: XIO(@de25fda7@.Flags.AFC_Set_Clock)LIM(1,@de25fda7@.CycleCounter,16)[ADD(6,8192,@de25fda7@.Meters[5].Variables.BID) ,XIO(@de25fda7@.EnableStatus.Meter6) [OTE(@de25fda7@.Meters[5].Variables.BID.8) ,OTU(@de25fda7@.DisableMeter.Meter6) ] ,XIC(@de25fda7@.EnableStatus.Meter6) OTU(@de25fda7@.EnableMeter.Meter6) ,XIO(@de25fda7@.Meters[5].Profile.MeterType) XIO(@de25fda7@.Meters[5].Profile.ProductGroup) COP(@de25fda7@.Meters[5].Variables.DifferentialGas.Temperature,@de25fda7@.outputbuffer[64],6) ,XIO(@de25fda7@.Meters[5].Profile.MeterType) XIC(@de25fda7@.Meters[5].Profile.ProductGroup) [COP(@de25fda7@.Meters[5].Variables.DifferentialLiquid.Water_Percent,@de25fda7@.outputbuffer[63],1) ,COP(@de25fda7@.Meters[5].Variables.DifferentialLiquid.Temperature,@de25fda7@.outputbuffer[64],8) ] ,XIC(@de25fda7@.Meters[5].Profile.MeterType) XIO(@de25fda7@.Meters[5].Profile.ProductGroup) [COP(@de25fda7@.Meters[5].Variables.LinearGas.Temperature,@de25fda7@.outputbuffer[64],4) ,COP(@de25fda7@.Meters[5].Variables.LinearGas.Meter_Pulses,@de25fda7@.outputbuffer[68],2) ,COP(@de25fda7@.Meters[5].Variables.LinearGas.Pulse_Frequency,@de25fda7@.outputbuffer[72],2) ] ,XIC(@de25fda7@.Meters[5].Profile.MeterType) XIC(@de25fda7@.Meters[5].Profile.ProductGroup) [COP(@de25fda7@.Meters[5].Variables.LinearLiquid.Water_Percent,@de25fda7@.outputbuffer[63],1) ,COP(@de25fda7@.Meters[5].Variables.LinearLiquid.Temperature,@de25fda7@.outputbuffer[64],4) ,COP(@de25fda7@.Meters[5].Variables.LinearLiquid.Meter_Pulses,@de25fda7@.outputbuffer[68],2) ,COP(@de25fda7@.Meters[5].Variables.LinearLiquid.Density,@de25fda7@.outputbuffer[70],4) ] ,MOV(@de25fda7@.Meters[5].Variables.BID,@de25fda7@.outputbuffer[62]) ];
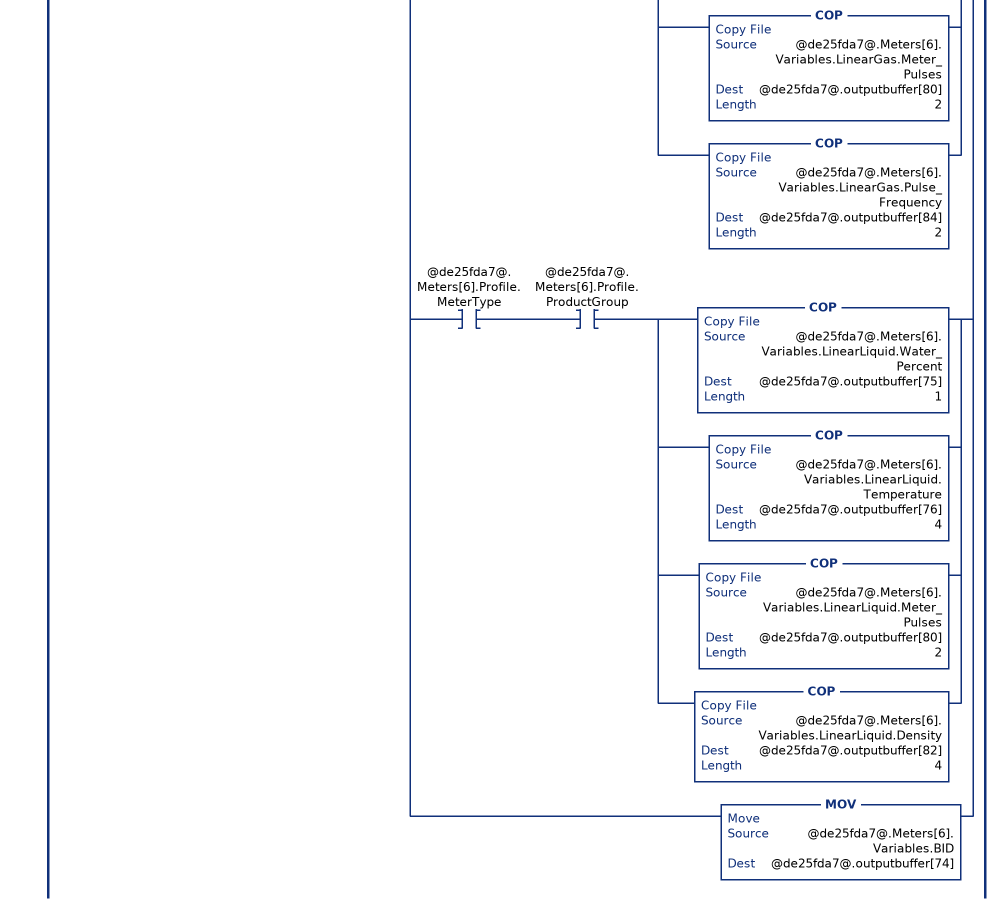
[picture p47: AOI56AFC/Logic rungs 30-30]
   30: XIO(@de25fda7@.Flags.AFC_Set_Clock)LIM(1,@de25fda7@.CycleCounter,16)[ADD(7,8192,@de25fda7@.Meters[6].Variables.BID) ,XIO(@de25fda7@.EnableStatus.Meter7) [OTE(@de25fda7@.Meters[6].Variables.BID.8) ,OTU(@de25fda7@.DisableMeter.Meter7) ] ,XIC(@de25fda7@.EnableStatus.Meter7) OTU(@de25fda7@.EnableMeter.Meter7) ,XIO(@de25fda7@.Meters[6].Profile.MeterType) XIO(@de25fda7@.Meters[6].Profile.ProductGroup) COP(@de25fda7@.Meters[6].Variables.DifferentialGas.Temperature,@de25fda7@.outputbuffer[76],6) ,XIO(@de25fda7@.Meters[6].Profile.MeterType) XIC(@de25fda7@.Meters[6].Profile.ProductGroup) [COP(@de25fda7@.Meters[6].Variables.DifferentialLiquid.Water_Percent,@de25fda7@.outputbuffer[75],1) ,COP(@de25fda7@.Meters[6].Variables.DifferentialLiquid.Temperature,@de25fda7@.outputbuffer[76],8) ] ,XIC(@de25fda7@.Meters[6].Profile.MeterType) XIO(@de25fda7@.Meters[6].Profile.ProductGroup) [COP(@de25fda7@.Meters[6].Variables.LinearGas.Temperature,@de25fda7@.outputbuffer[76],4) ,COP(@de25fda7@.Meters[6].Variables.LinearGas.Meter_Pulses,@de25fda7@.outputbuffer[80],2) ,COP(@de25fda7@.Meters[6].Variables.LinearGas.Pulse_Frequency,@de25fda7@.outputbuffer[84],2) ] ,XIC(@de25fda7@.Meters[6].Profile.MeterType) XIC(@de25fda7@.Meters[6].Profile.ProductGroup) [COP(@de25fda7@.Meters[6].Variables.LinearLiquid.Water_Percent,@de25fda7@.outputbuffer[75],1) ,COP(@de25fda7@.Meters[6].Variables.LinearLiquid.Temperature,@de25fda7@.outputbuffer[76],4) ,COP(@de25fda7@.Meters[6].Variables.LinearLiquid.Meter_Pulses,@de25fda7@.outputbuffer[80],2) ,COP(@de25fda7@.Meters[6].Variables.LinearLiquid.Density,@de25fda7@.outputbuffer[82],4) ] ,MOV(@de25fda7@.Meters[6].Variables.BID,@de25fda7@.outputbuffer[74]) ];
